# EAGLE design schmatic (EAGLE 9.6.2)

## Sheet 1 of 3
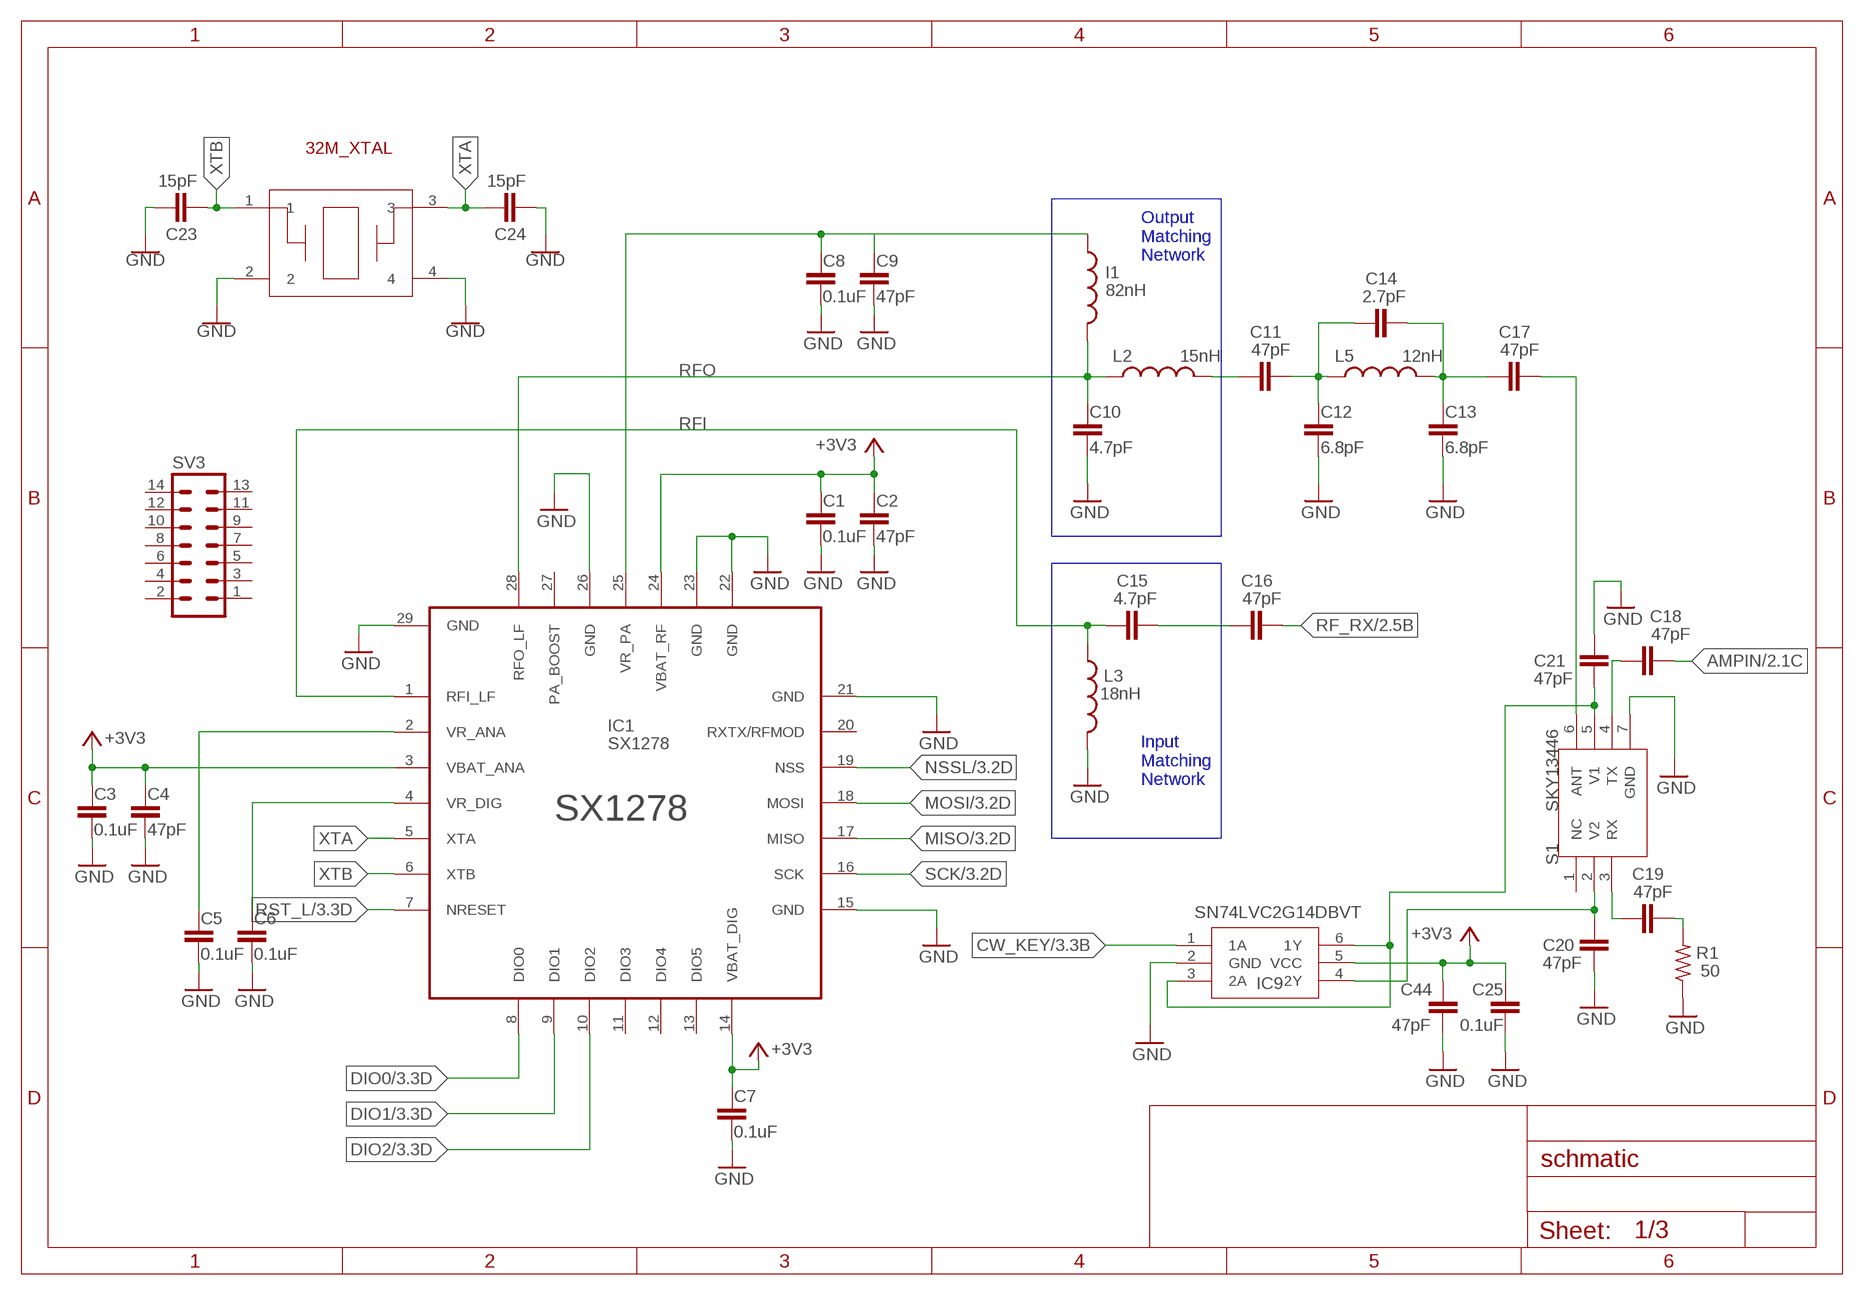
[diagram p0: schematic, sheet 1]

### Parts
C1  0.1uF  CAPACITOR  [M(1005)_US(0402)]
C2  47pF  CAPACITOR  [M(1005)_US(0402)]
C3  0.1uF  CAPACITOR  [M(1005)_US(0402)]
C4  47pF  CAPACITOR  [M(1005)_US(0402)]
C5  0.1uF  CAPACITOR  [M(1005)_US(0402)]
C6  0.1uF  CAPACITOR  [M(1005)_US(0402)]
C7  0.1uF  CAPACITOR  [M(1005)_US(0402)]
C8  0.1uF  CAPACITOR  [M(1005)_US(0402)]
C9  47pF  CAPACITOR  [M(1005)_US(0402)]
C10  4.7pF  CAPACITOR  [M(1005)_US(0402)]
C11  47pF  CAPACITOR  [M(1005)_US(0402)]
C12  6.8pF  CAPACITOR  [M(1005)_US(0402)]
C13  6.8pF  CAPACITOR  [M(1005)_US(0402)]
C14  2.7pF  CAPACITOR  [M(1005)_US(0402)]
C15  4.7pF  CAPACITOR  [M(1005)_US(0402)]
C16  47pF  CAPACITOR  [M(1005)_US(0402)]
C17  47pF  CAPACITOR  [M(1005)_US(0402)]
C18  47pF  CAPACITOR  [M(1005)_US(0402)]
C19  47pF  CAPACITOR  [M(1005)_US(0402)]
C20  47pF  CAPACITOR  [M(1005)_US(0402)]
C21  47pF  CAPACITOR  [M(1005)_US(0402)]
C23  15pF  CAP_(M1005)_0402  [CAP_(M1005)_0402]
C24  15pF  CAP_(M1005)_0402  [CAP_(M1005)_0402]
C25  0.1uF  CAPACITOR  [M(1005)_US(0402)]
C44  47pF  CAPACITOR  [M(1005)_US(0402)]
I1  82nH  INDUCTOR1608  [M(1608)_US(0603)]
IC1  SX1278  [SX1278]
IC9  SN74LVC2G14DBVT  SN74LVC2G34DBVR  [SOT-23-6]
L2  15nH  INDUCTOR  [M(1005)_US(0402)]
L3  18nH  INDUCTOR  [M(1005)_US(0402)]
L5  12nH  INDUCTOR  [M(1005)_US(0402)]
Q1  NX2520SA-32MHZ  [NX2520SA]
R1  50  RESISTOR1608  [M(1608)_US(0603)]
S1  SKY13446  [SKY13446]
SV3  ML14  [ML14]

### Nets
+3V1: C5.1 IC1.2(VR_ANA)
+3V2: C6.1 IC1.4(VR_DIG)
+3V3: C1.1 C2.1 C3.1 C4.1 C7.1 C25.1 C44.1 IC1.3(VBAT_ANA) IC1.14(VBAT_DIG) IC1.24(VBAT_RF) IC9.5(VCC) ; also sheet 2,3
+3V4: C8.1 C9.1 I1.1 IC1.25(VR_PA)
AMPIN: C18.2 ; also sheet 2
CW_KEY: IC9.1(1A) ; also sheet 3
DIO0: IC1.8(DIO0) ; also sheet 3
DIO1: IC1.9(DIO1) ; also sheet 3
DIO2: IC1.10(DIO2) ; also sheet 3
GND: C1.2 C2.2 C3.2 C4.2 C5.2 C6.2 C7.2 C8.2 C9.2 C10.2 C12.2 C13.2 C20.1 C21.2 C23.1 C24.2 C25.2 C44.2 IC1.15(GND) IC1.21(GND) IC1.22(GND) IC1.23(GND) IC1.26(GND) IC1.29(GND) IC9.2(GND) L3.2 Q1.2 Q1.4 R1.1 S1.7(GND) ; also sheet 2,3
MISO: IC1.17(MISO) ; also sheet 3
MOSI: IC1.18(MOSI) ; also sheet 3
N$1: C11.1 L2.2
N$2: C11.2 C12.1 C14.1 L5.1
N$3: C13.1 C14.2 C17.1 L5.2
N$4: C17.2 S1.6(ANT)
N$5: C15.2 C16.1
N$6: C18.1 S1.4(TX)
N$7: C19.1 S1.3(RX)
N$8: C19.2 R1.2
N$11: C20.2 IC9.4(2Y) S1.2(V2)
N$27: C21.1 IC9.3(2A) IC9.6(1Y) S1.5(V1)
NSSL: IC1.19(NSS) ; also sheet 3
RF_RX: C16.2 ; also sheet 2
RFI: C15.1 IC1.1(RFI_LF) L3.1
RFO: C10.1 I1.2 IC1.28(RFO_LF) L2.1
RST_L: IC1.7(NRESET) ; also sheet 3
SCK: IC1.16(SCK) ; also sheet 3
XTA: C24.1 IC1.5(XTA) Q1.3
XTB: C23.2 IC1.6(XTB) Q1.1
Unconnected: IC1.11(DIO3) IC1.12(DIO4) IC1.13(DIO5) IC1.20(RXTX/RFMOD) IC1.27(PA_BOOST) S1.1(NC) SV3.1 SV3.2 SV3.3 SV3.4 SV3.5 SV3.6 SV3.7 SV3.8 SV3.9 SV3.10 SV3.11 SV3.12 SV3.13 SV3.14

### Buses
B$1
B$2

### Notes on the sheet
- 32M_XTAL
- Output
  Matching
  Network
- Input
  Matching
  Network

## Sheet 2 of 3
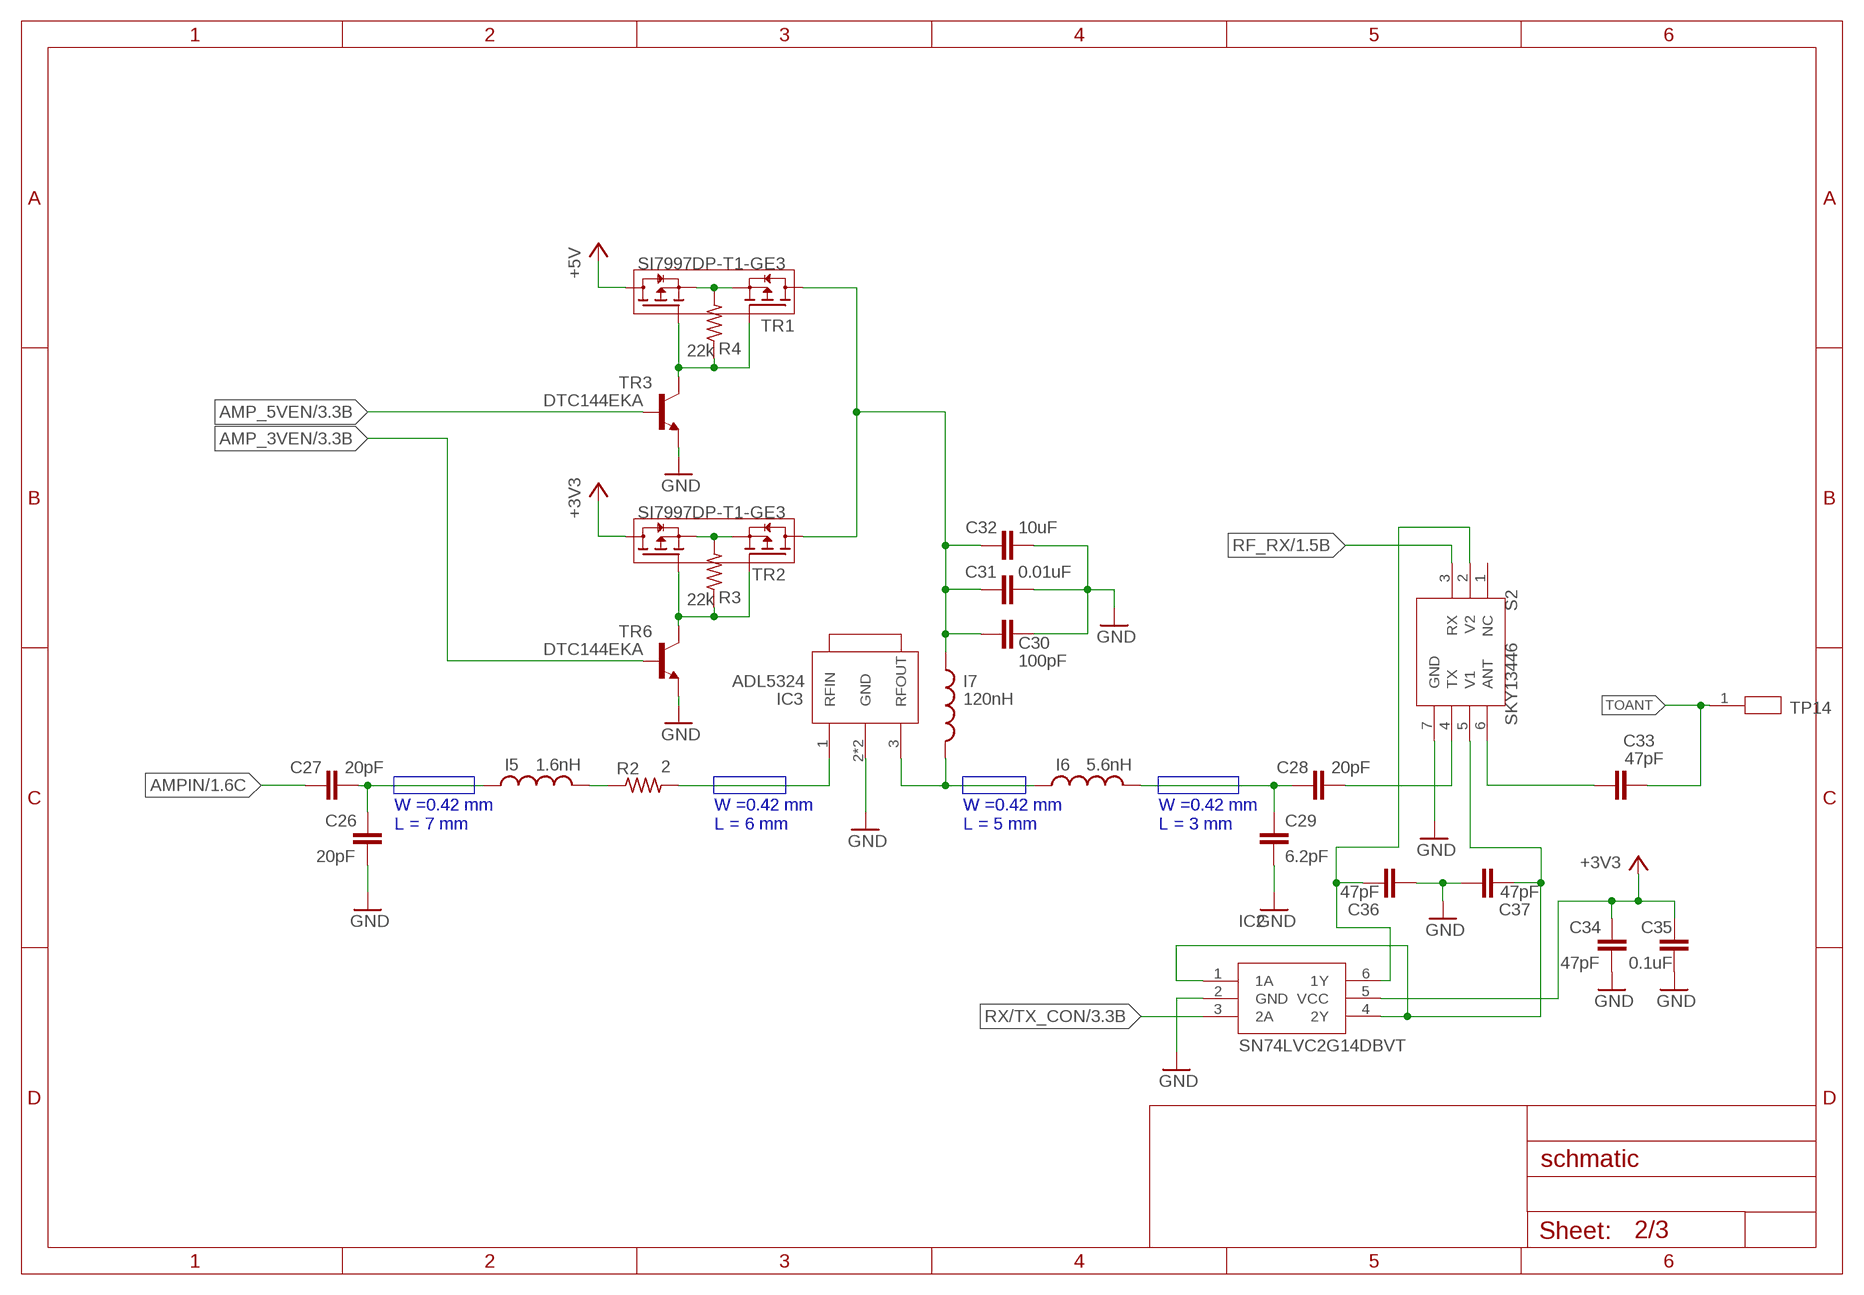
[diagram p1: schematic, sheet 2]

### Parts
C26  20pF  CAPACITOR  [M(1005)_US(0402)]
C27  20pF  CAPACITOR  [M(1005)_US(0402)]
C28  20pF  CAPACITOR  [M(1005)_US(0402)]
C29  6.2pF  CAPACITOR  [M(1005)_US(0402)]
C30  100pF  CAPACITOR  [M(1005)_US(0402)]
C31  0.01uF  CAPACITOR  [M(1005)_US(0402)]
C32  10uF  CAPACITOR1608  [M(1608)_US(0603)]
C33  47pF  CAPACITOR  [M(1005)_US(0402)]
C34  47pF  CAPACITOR  [M(1005)_US(0402)]
C35  0.1uF  CAPACITOR  [M(1005)_US(0402)]
C36  47pF  CAPACITOR  [M(1005)_US(0402)]
C37  47pF  CAPACITOR  [M(1005)_US(0402)]
I5  1.6nH  INDUCTOR  [M(1005)_US(0402)]
I6  5.6nH  INDUCTOR  [M(1005)_US(0402)]
I7  120nH  INDUCTOR2012  [M(2012)_US(0805)]
IC2  SN74LVC2G14DBVT  SN74LVC2G34DBVR  [SOT-23-6]
IC3  ADL5324  [ADL5324]
R2  2  RESISTOR1608  [M(1608)_US(0603)]
R3  22k  RESISTOR1608  [M(1608)_US(0603)]
R4  22k  RESISTOR1608  [M(1608)_US(0603)]
S2  SKY13446  [SKY13446]
TP14  TEST_POINT  [TEST_POINT_1.5MM]
TR1  SI7997DP-T1-GE3  [SI7997DP-T1-GE3]
TR2  SI7997DP-T1-GE3  [SI7997DP-T1-GE3]
TR3  DTC144EKA  [SOT346-R]
TR6  DTC144EKA  [SOT346-R]

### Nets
+3V3: C34.1 C35.1 IC2.5(VCC) TR2.7(D1) TR2.8(D1) TR2.10(D1) ; also sheet 1,3
+3V5: C30.1
+5V: TR1.7(D1) TR1.8(D1) TR1.10(D1) ; also sheet 3
AMP_3VEN: TR6.2(B) ; also sheet 3
AMP_5VEN: TR3.2(B) ; also sheet 3
AMPIN: C27.1 ; also sheet 1
AMPPWR: C30.2 C31.2 C32.1 I7.1 TR1.5(D2) TR1.6(D2) TR1.9(D2) TR2.5(D2) TR2.6(D2) TR2.9(D2)
GND: C26.2 C29.2 C31.1 C32.2 C34.2 C35.2 C36.1 C37.2 IC2.2(GND) IC3.2(GND) IC3.4(GND) S2.7(GND) TR3.1(E) TR6.1(E) ; also sheet 1,3
N$9: C26.1 C27.2 I5.1
N$10: C37.1 IC2.1(1A) IC2.4(2Y) S2.5(V1)
N$12: I5.2 R2.1
N$13: IC3.1(RFIN) R2.2
N$14: I6.1 I7.2 IC3.3(RFOUT)
N$15: C28.1 C29.1 I6.2
N$16: C28.2 S2.4(TX)
N$17: C33.1 S2.6(ANT)
N$18: R4.2 TR1.1(S1) TR1.3(S2)
N$19: R3.2 TR2.1(S1) TR2.3(S2)
N$20: C36.2 IC2.6(1Y) S2.2(V2)
N$22: R4.1 TR1.2(G1) TR1.4(G2) TR3.3(C)
N$23: R3.1 TR2.2(G1) TR2.4(G2) TR6.3(C)
RF_RX: S2.3(RX) ; also sheet 1
RX/TX_CON: IC2.3(2A) ; also sheet 3
TOANT: C33.2 TP14.1
Unconnected: S2.1(NC)

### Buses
B$3
B$4
B$5
B$6

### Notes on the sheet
- W =0.42 mm
  L = 7 mm
- W =0.42 mm
  L = 6 mm
- W =0.42 mm
  L = 5 mm
- W =0.42 mm
  L = 3 mm

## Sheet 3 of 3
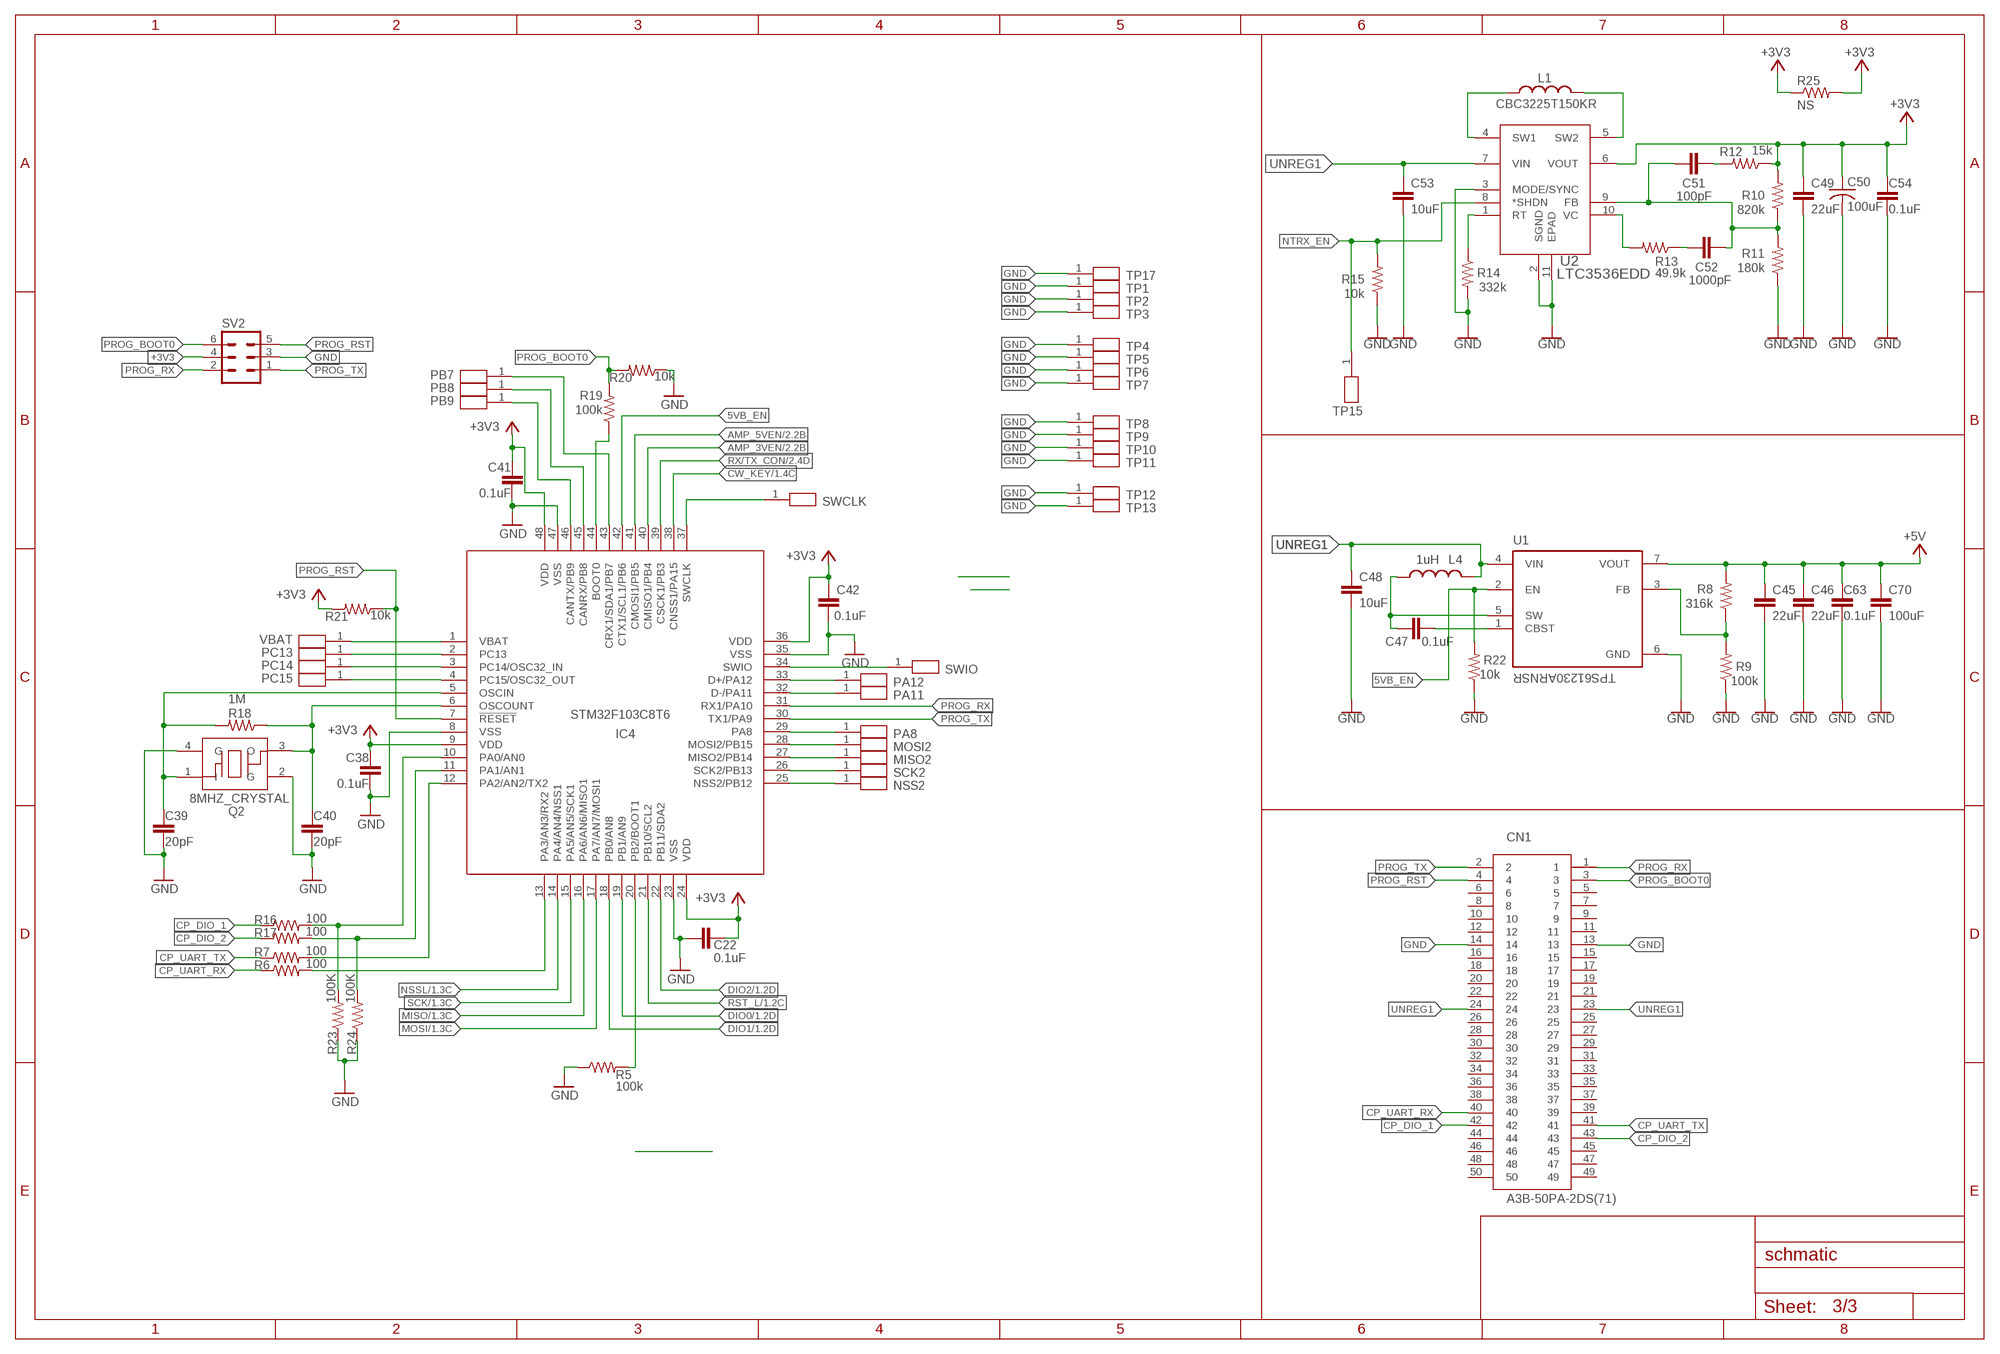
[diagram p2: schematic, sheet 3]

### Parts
C22  0.1uF  CAPACITOR  [M(1005)_US(0402)]
C38  0.1uF  CAPACITOR  [M(1005)_US(0402)]
C39  20pF  CAPACITOR  [M(1005)_US(0402)]
C40  20pF  CAPACITOR  [M(1005)_US(0402)]
C41  0.1uF  CAPACITOR  [M(1005)_US(0402)]
C42  0.1uF  CAPACITOR  [M(1005)_US(0402)]
C45  22uF  CAPACITOR1608  [M(1608)_US(0603)]
C46  22uF  CAPACITOR1608  [M(1608)_US(0603)]
C47  0.1uF  CAPACITOR  [M(1005)_US(0402)]
C48  10uF  CAPACITOR1608  [M(1608)_US(0603)]
C49  22uF  CAPACITOR1608  [M(1608)_US(0603)]
C50  100uF  C-USC1210  [C1210]
C51  100pF  CAPACITOR  [M(1005)_US(0402)]
C52  1000pF  CAPACITOR  [M(1005)_US(0402)]
C53  10uF  CAPACITOR1608  [M(1608)_US(0603)]
C54  0.1uF  CAPACITOR  [M(1005)_US(0402)]
C63  0.1uF  CAPACITOR  [M(1005)_US(0402)]
C70  100uF  CAPACITOR2012  [M(2012)_US(0805)]
CN1  A3B-50PA-2DS(71)  [A3B-50PA-2DS(71)]
IC4  STM32F103C8T6  [STM32F103C8T6]
L1  CBC3225T150KR  INDUCTOR3225  [M(3225)_US(1210)]
L4  1uH  AMDLA3020S-1R5MT  [AMDLA3020S-1R5MT]
MISO2  TEST_POINT  [TEST_POINT_1.5MM]
MOSI2  TEST_POINT  [TEST_POINT_1.5MM]
NSS2  TEST_POINT  [TEST_POINT_1.5MM]
PA8  TEST_POINT  [TEST_POINT_1.5MM]
PA11  TEST_POINT  [TEST_POINT_1.5MM]
PA12  TEST_POINT  [TEST_POINT_1.5MM]
PB7  TEST_POINT  [TEST_POINT_1.5MM]
PB8  TEST_POINT  [TEST_POINT_1.5MM]
PB9  TEST_POINT  [TEST_POINT_1.5MM]
PC13  TEST_POINT  [TEST_POINT_1.5MM]
PC14  TEST_POINT  [TEST_POINT_1.5MM]
PC15  TEST_POINT  [TEST_POINT_1.5MM]
Q2  8MHZ_CRYSTAL  [ECS-80-18-30B-JEM-TR]
R5  100k  RESISTOR  [M(1005)_US(0402)]
R6  100  RESISTOR  [M(1005)_US(0402)]
R7  100  RESISTOR  [M(1005)_US(0402)]
R8  316k  RESISTOR1608  [M(1608)_US(0603)]
R9  100k  RESISTOR1608  [M(1608)_US(0603)]
R10  820k  RESISTOR1608  [M(1608)_US(0603)]
R11  180k  RESISTOR1608  [M(1608)_US(0603)]
R12  15k  RESISTOR1608  [M(1608)_US(0603)]
R13  49.9k  RESISTOR1608  [M(1608)_US(0603)]
R14  332k  RESISTOR1608  [M(1608)_US(0603)]
R15  10k  RESISTOR  [M(1005)_US(0402)]
R16  100  RESISTOR  [M(1005)_US(0402)]
R17  100  RESISTOR  [M(1005)_US(0402)]
R18  1M  RESISTOR1608  [M(1608)_US(0603)]
R19  100k  RESISTOR  [M(1005)_US(0402)]
R20  10k  RESISTOR  [M(1005)_US(0402)]
R21  10k  RESISTOR  [M(1005)_US(0402)]
R22  10k  RESISTOR  [M(1005)_US(0402)]
R23  100K  RESISTOR  [M(1005)_US(0402)]
R24  100K  RESISTOR  [M(1005)_US(0402)]
R25  NS  RESISTOR2012  [M(2012)_US(0805)]
SCK2  TEST_POINT  [TEST_POINT_1.5MM]
SV2  MA03-2  [MA03-2]
SWCLK  TEST_POINT  [TEST_POINT_1.5MM]
SWIO  TEST_POINT  [TEST_POINT_1.5MM]
TP1  TEST_POINT  [TEST_POINT_1.5MM]
TP2  TEST_POINT  [TEST_POINT_1.5MM]
TP3  TEST_POINT  [TEST_POINT_1.5MM]
TP4  TEST_POINT  [TEST_POINT_1.5MM]
TP5  TEST_POINT  [TEST_POINT_1.5MM]
TP6  TEST_POINT  [TEST_POINT_1.5MM]
TP7  TEST_POINT  [TEST_POINT_1.5MM]
TP8  TEST_POINT  [TEST_POINT_1.5MM]
TP9  TEST_POINT  [TEST_POINT_1.5MM]
TP10  TEST_POINT  [TEST_POINT_1.5MM]
TP11  TEST_POINT  [TEST_POINT_1.5MM]
TP12  TEST_POINT  [TEST_POINT_1.5MM]
TP13  TEST_POINT  [TEST_POINT_1.5MM]
TP15  TEST_POINT  [TEST_POINT_1.5MM]
TP17  TEST_POINT  [TEST_POINT_1.5MM]
U1  TPS61230ARNSR  [IC_TPS61230ARNSR]
U2  LTC3536EDD  LTC3536EDD#TRPBF  [DFN-10_DD]
VBAT  TEST_POINT  [TEST_POINT_1.5MM]

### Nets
5VB_EN: IC4.42(CTX1/SCL1/PB6) R22.2 U1.2(EN)
+3V3: C22.1 C38.1 C41.1 C42.1 C49.1 C50.1 C54.1 IC4.9(VDD) IC4.24(VDD) IC4.36(VDD) IC4.48(VDD) R10.2 R12.1 R21.2 R25.1 R25.2 SV2.4 U2.6(VOUT) ; also sheet 1,2
+5V: C45.1 C46.1 C63.1 C70.1 R8.2 U1.7(VOUT) ; also sheet 2
AMP_3VEN: IC4.40(CMISO1/PB4) ; also sheet 2
AMP_5VEN: IC4.41(CMOSI1/PB5) ; also sheet 2
C_UART_RX: IC4.13(PA3/AN3/RX2) R6.2
C_UART_TX: IC4.12(PA2/AN2/TX2) R7.2
CP_DIO_1: CN1.42 R16.1
CP_DIO_2: CN1.43 R17.1
CP_UART_RX: CN1.40 R6.1
CP_UART_TX: CN1.41 R7.1
CW_KEY: IC4.38(CNSS1/PA15) ; also sheet 1
DIO0: IC4.19(PB1/AN9) ; also sheet 1
DIO1: IC4.18(PB0/AN8) ; also sheet 1
DIO2: IC4.22(PB11/SDA2) ; also sheet 1
GND: C22.2 C38.2 C39.2 C40.2 C41.2 C42.2 C45.2 C46.2 C48.2 C49.2 C50.2 C53.2 C54.2 C63.2 C70.2 CN1.13 CN1.14 IC4.8(VSS) IC4.23(VSS) IC4.35(VSS) IC4.47(VSS) Q2.2(G) Q2.4(G) R5.1 R9.1 R11.1 R14.2 R15.1 R20.1 R22.1 R23.1 R24.1 SV2.3 TP1.1 TP2.1 TP3.1 TP4.1 TP5.1 TP6.1 TP7.1 TP8.1 TP9.1 TP10.1 TP11.1 TP12.1 TP13.1 TP17.1 U1.6(GND) U2.2(SGND) U2.3(MODE/SYNC) U2.11(EPAD) ; also sheet 1,2
MISO: IC4.16(PA6/AN6/MISO1) ; also sheet 1
MOSI: IC4.17(PA7/AN7/MOSI1) ; also sheet 1
N$24: IC4.10(PA0/AN0) R16.2 R23.2
N$25: IC4.20(PB2/BOOT1) R5.2
N$26: IC4.11(PA1/AN1) R17.2 R24.2
N$28: C39.1 IC4.5(OSCIN) Q2.1(I) R18.2
N$29: C40.1 IC4.6(OSCOUNT) Q2.3(O) R18.1
N$30: L1.1 U2.4(SW1)
N$31: R8.1 R9.2 U1.3(FB)
N$32: C47.1 L4.1 U1.5(SW)
N$33: L1.2 U2.5(SW2)
N$34: C47.2 U1.1(CBST)
N$35: IC4.1(VBAT) VBAT.1
N$36: C51.2 R12.2
N$37: C51.1 C52.2 R10.1 R11.2 U2.9(FB)
N$38: IC4.44(BOOT0) R19.1
N$39: C52.1 R13.1
N$40: R13.2 U2.10(VC)
N$41: R14.1 U2.1(RT)
N$42: IC4.4(PC15/OSC32_OUT) PC15.1
N$44: IC4.3(PC14/OSC32_IN) PC14.1
N$45: IC4.2(PC13) PC13.1
N$46: IC4.27(MISO2/PB14) MISO2.1
N$47: IC4.28(MOSI2/PB15) MOSI2.1
N$48: IC4.33(D+/PA12) PA12.1
N$49: IC4.32(D-/PA11) PA11.1
N$50: IC4.29(PA8) PA8.1
N$68: IC4.26(SCK2/PB13) SCK2.1
N$69: IC4.25(NSS2/PB12) NSS2.1
NSSL: IC4.14(PA4/AN4/NSS1) ; also sheet 1
NTRX_EN: R15.2 TP15.1 U2.8(*SHDN)
PB7: IC4.43(CRX1/SDA1/PB7) PB7.1
PB8: IC4.45(CANRX/PB8) PB8.1
PB9: IC4.46(CANTX/PB9) PB9.1
PROG_BOOT0: CN1.3 R19.2 R20.2 SV2.6
PROG_RST: CN1.4 IC4.7(!RESET) R21.1 SV2.5
PROG_RX: CN1.1 IC4.31(RX1/PA10) SV2.2
PROG_TX: CN1.2 IC4.30(TX1/PA9) SV2.1
RST_L: IC4.21(PB10/SCL2) ; also sheet 1
RX/TX_CON: IC4.39(CSCK1/PB3) ; also sheet 2
SCK: IC4.15(PA5/AN5/SCK1) ; also sheet 1
SWCLK: IC4.37(SWCLK) SWCLK.1
SWIO: IC4.34(SWIO) SWIO.1
UNREG1: C48.1 C53.1 CN1.23 CN1.24 L4.2 U1.4(VIN) U2.7(VIN)
Unconnected: CN1.5 CN1.6 CN1.7 CN1.8 CN1.9 CN1.10 CN1.11 CN1.12 CN1.15 CN1.16 CN1.17 CN1.18 CN1.19 CN1.20 CN1.21 CN1.22 CN1.25 CN1.26 CN1.27 CN1.28 CN1.29 CN1.30 CN1.31 CN1.32 CN1.33 CN1.34 CN1.35 CN1.36 CN1.37 CN1.38 CN1.39 CN1.44 CN1.45 CN1.46 CN1.47 CN1.48 CN1.49 CN1.50

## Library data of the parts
C1-C22 C25-C42 C44-C49 C51-C54 C63 C70 = Tharindu_lib:CAPACITOR
C23 C24 = Tharindu:CAP_(M1005)_0402
C50 = adafruit:C-US: CAPACITOR, American symbol
CN1 = Tharindu1:A3B-50PA-2DS(71)
I1 I5-I7 L1-L3 L5 = Tharindu_lib:INDUCTOR
IC1 = Tharindu:SX1278
IC2 IC9 = Tharindu:SN74LVC2G34DBVR
IC3 = Tharindu:ADL5324
IC4 = Tharindu:STM32F103C8T6
L4 = Tharindu:AMDLA3020S-1R5MT
MISO2 MOSI2 NSS2 PA8 PA11 PA12 PB7-PB9 PC13-PC15 SCK2 SWCLK SWIO TP1-TP15 TP17 VBAT = Tharindu:TEST_POINT
Q1 = Tharindu:NX2520SA-32MHZ
Q2 = Tharindu:8MHZ_CRYSTAL
R1-R25 = Tharindu_lib:RESISTOR
S1 S2 = Tharindu:SKY13446
SV2 = con-lstb:MA03-2: PIN HEADER; OC_FARNELL: unknown; OC_NEWARK: unknown
SV3 = con-ml:ML14: HARTING; OC_FARNELL: unknown; OC_NEWARK: unknown
TR1 TR2 = Tharindu:SI7997DP-T1-GE3
TR3 TR6 = BIRDS3_CAM_MSN:DTC144EKA
U1 = TPS61230ARNSR:TPS61230ARNSR: Boost Switching Regulator IC Positive Adjustable 2.5V 1 Output 6A (Switch) 7-VFQFN Check availability; AVAILABILITY: In Stock; DESCRIPTION: 5-V/6-A High Efficiency Step-Up Converter in 2.0-mm x 2.0-mm QFN Package; MF: Texas Instruments; MP: TPS61230ARNSR; PACKAGE: VQFN-HR-7 Texas Instruments; PRICE: None; PURCHASE-URL: https://pricing.snapeda.com/search/part/TPS61230ARNSR/?ref=eda
U2 = LTC3536EDD_TRPBF:LTC3536EDD#TRPBF: Check availability; AVAILABILITY: In Stock; DESCRIPTION: 1A Low Noise, Buck-Boost DC/DC Converter; MF: Analog Devices; MP: LTC3536EDD#TRPBF; PACKAGE: DFN -10 Analog Devices; PRICE: None; PURCHASE-URL: https://pricing.snapeda.com/search/part/LTC3536EDD#TRPBF/?ref=eda

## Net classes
0 default: width 0.203 mm, drill 0.33 mm, clearance 0.203 mm
2 gnd: width 0.305 mm, drill 0.33 mm, clearance 0.203 mm
3 power usb: width 0.508 mm, drill 0.33 mm, clearance 0.203 mm

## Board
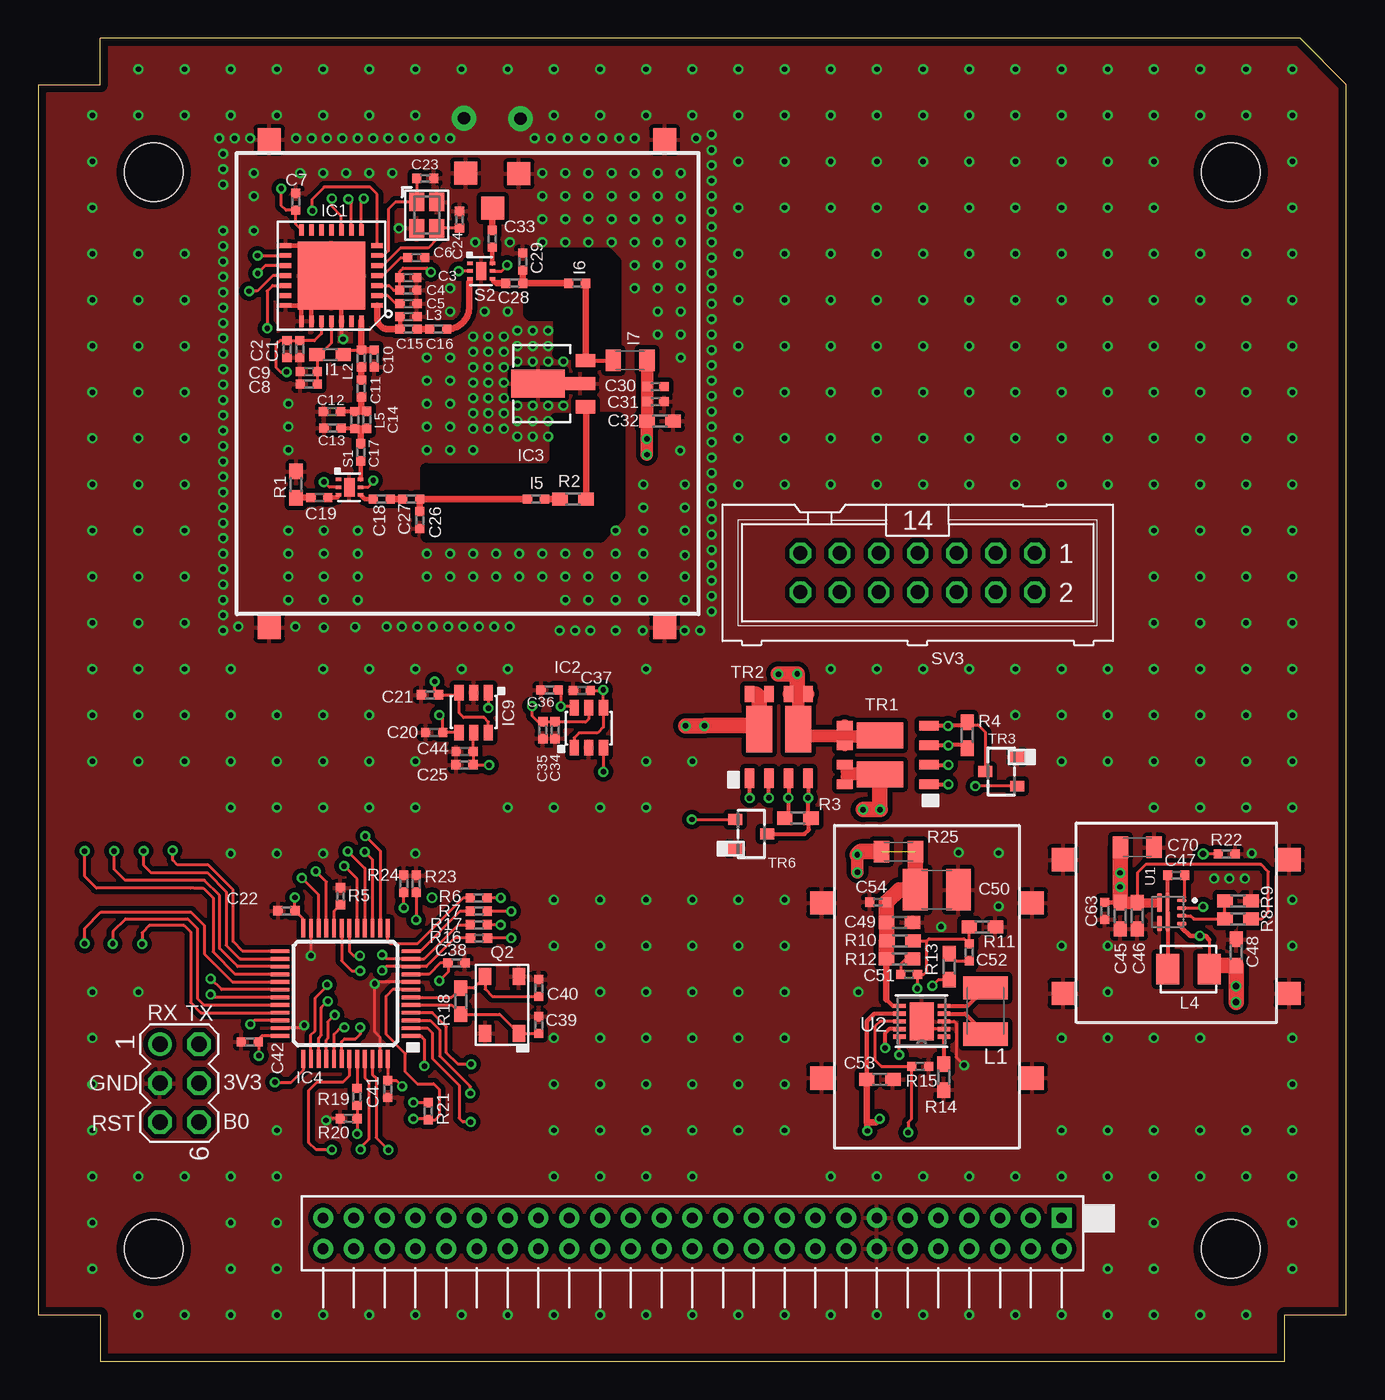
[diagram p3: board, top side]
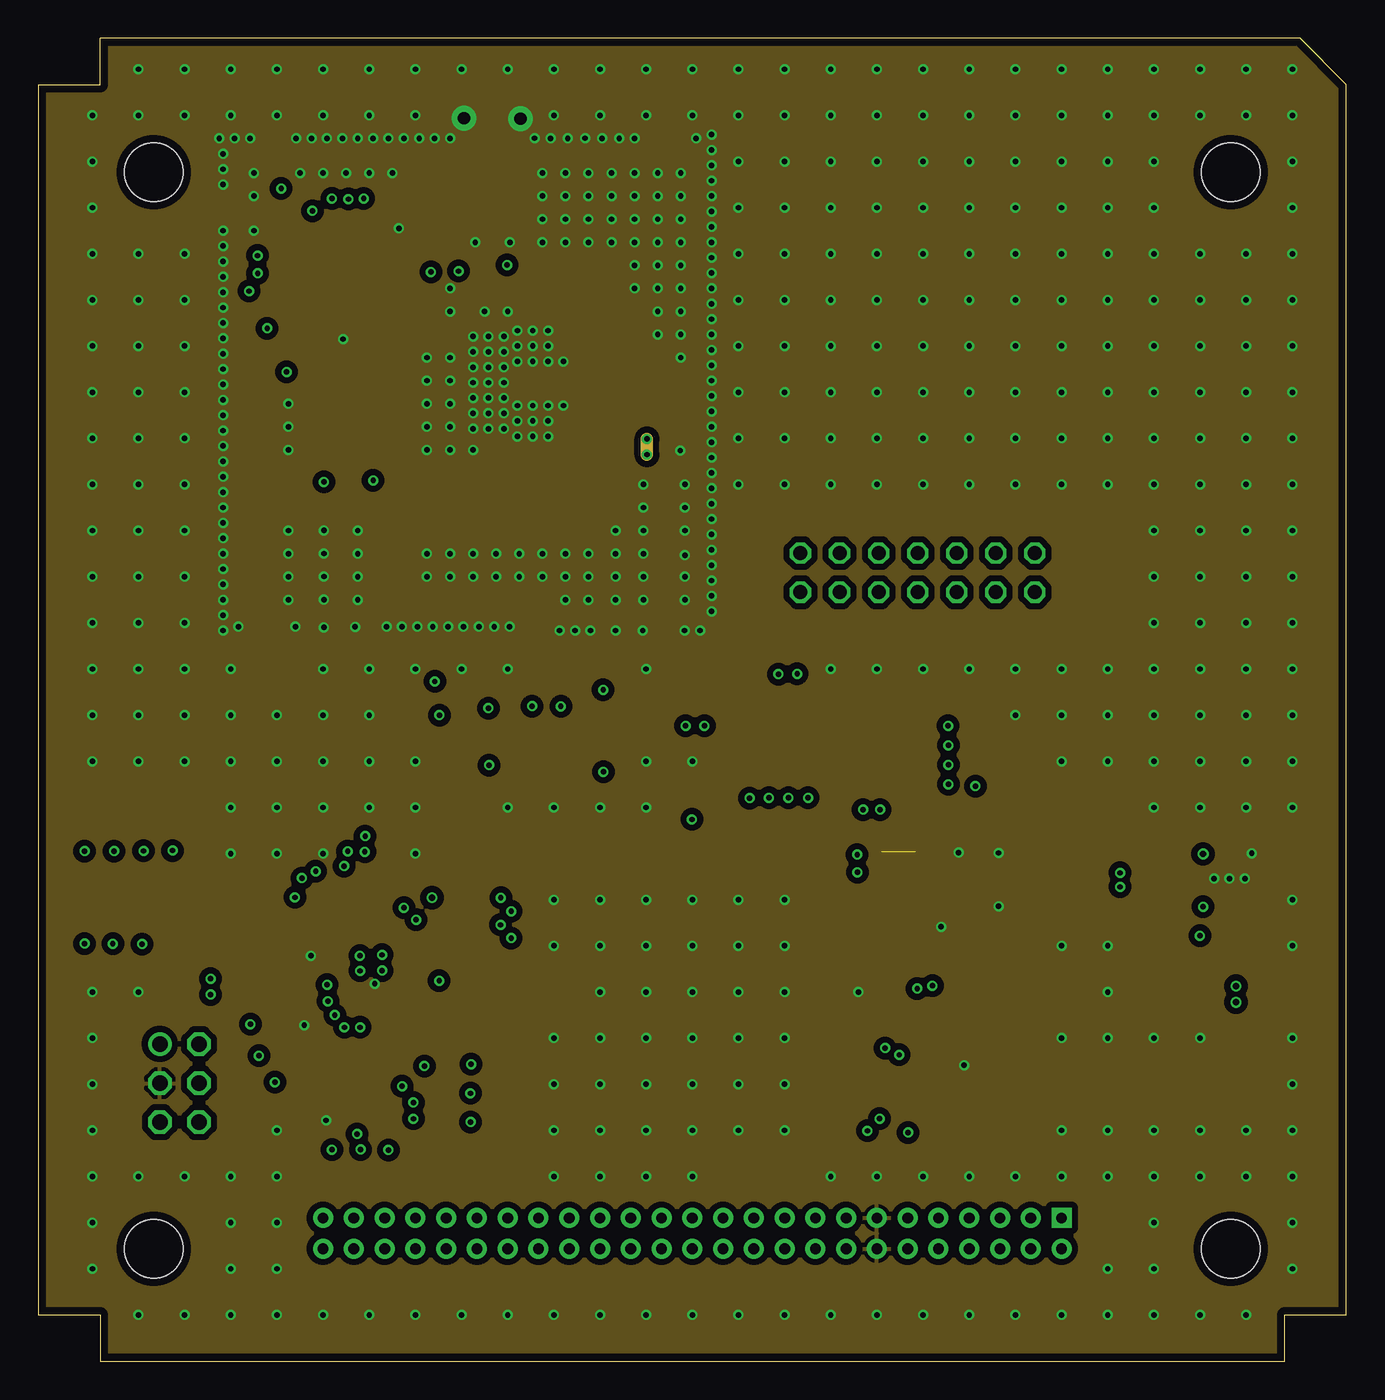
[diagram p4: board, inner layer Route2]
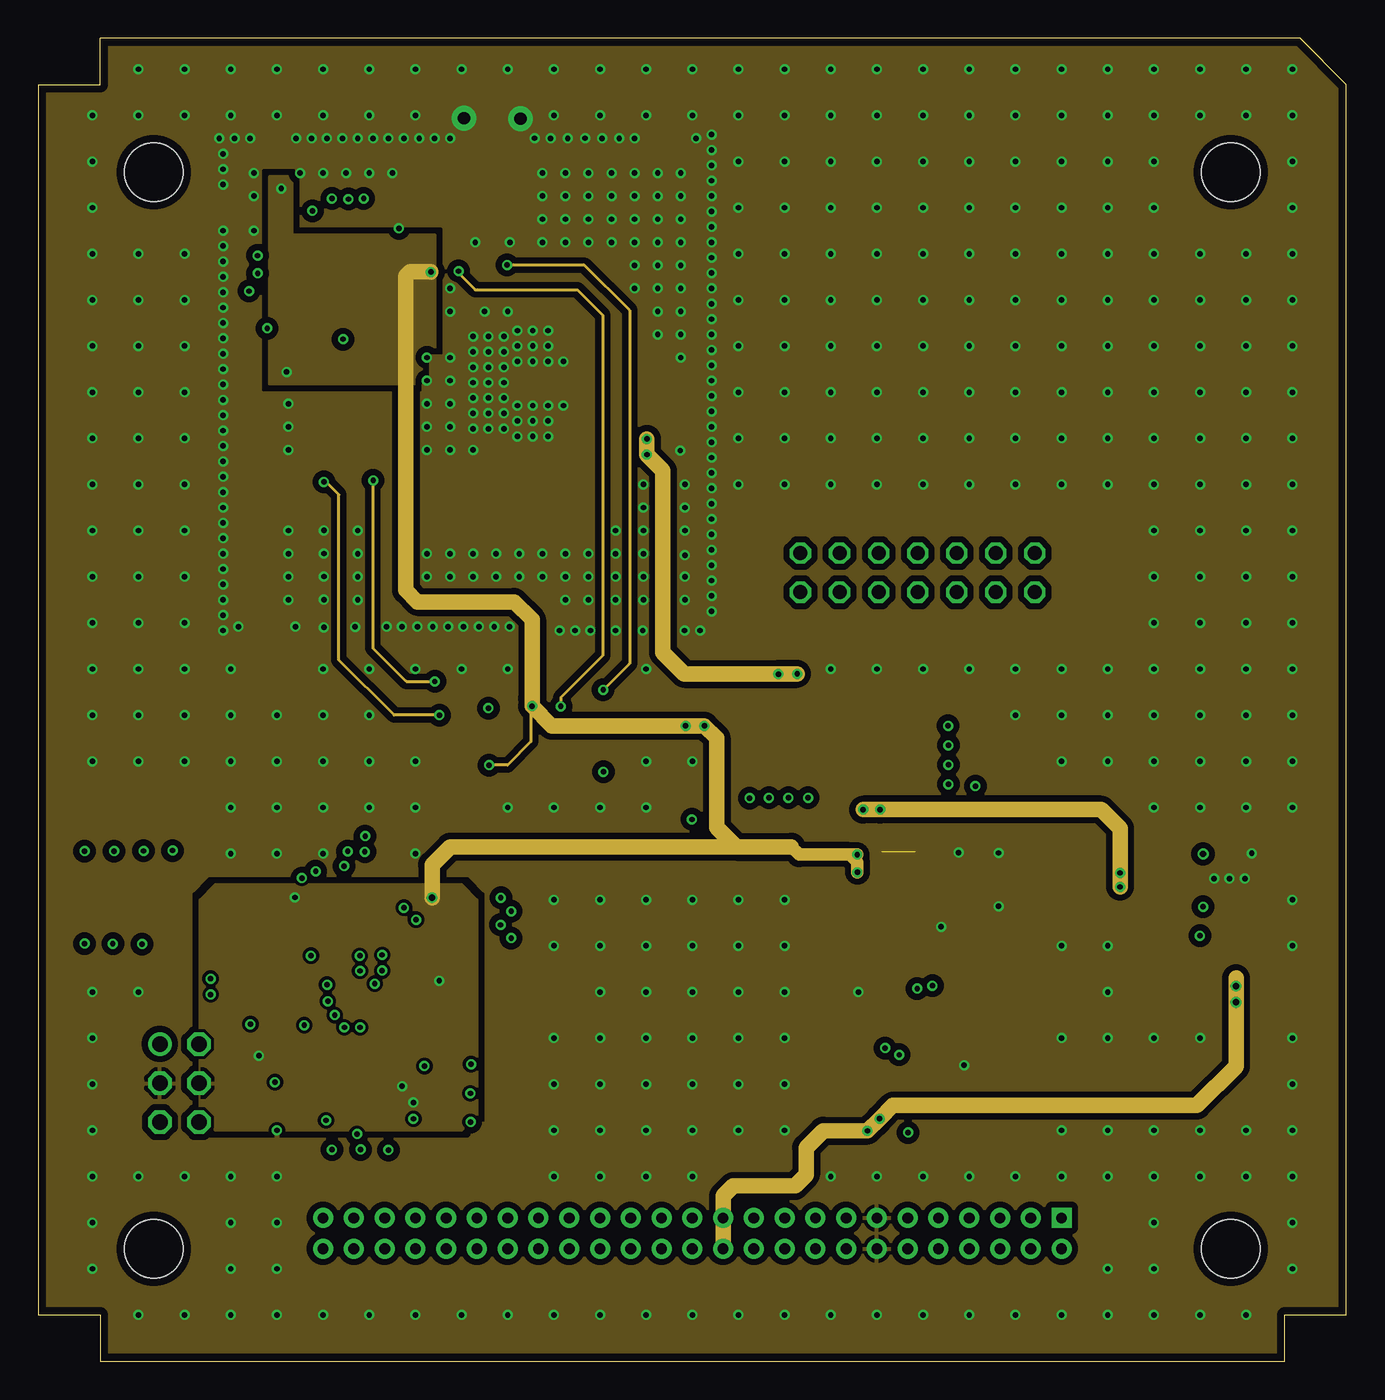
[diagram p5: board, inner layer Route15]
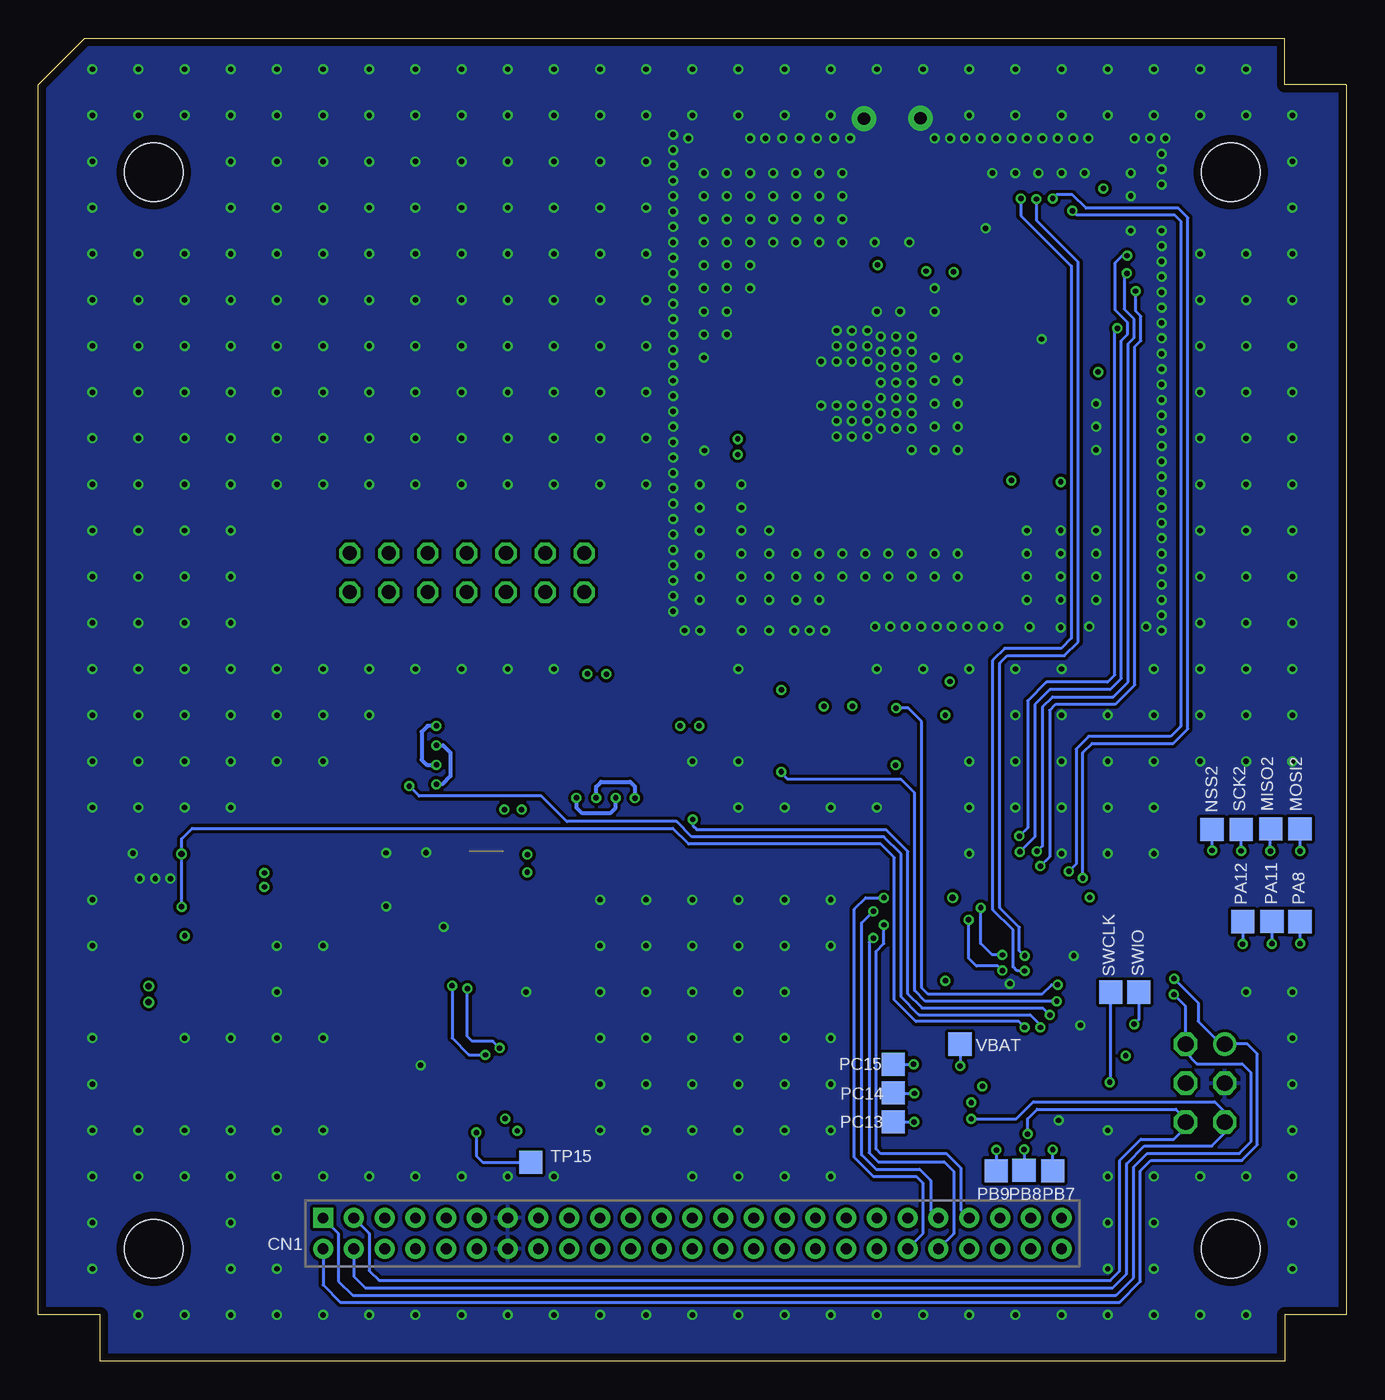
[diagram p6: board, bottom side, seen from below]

Size 85 x 86 mm. Coordinates in mm from the lower left corner, seen from the top.
Outline: 4,0 81,0 81,3 85,3 85,83 82,86 4,86 4,83 0,83 0,3 4,3 4,0
Copper layers (1+2*15+16): Top 0.018mm / dielectric 0.25mm / Route2 0.035mm / dielectric 1mm / Route15 0.035mm / dielectric 0.25mm / Bottom 0.018mm
Design rules "pban_5mil-l4": minimum track width 5mil, minimum drill 0.3mm, track to track 5mil, track to pad 0.229mm, pad to pad 5mil, via to via 5mil, smd to smd 5mil, copper to edge 0.5mm, drill to drill 0.5mm, minimum pad ring 0.15mm, minimum via ring 0.15mm, stop-mask expansion 4mil, vias tented up to drill 0.35mm, thermal gap 10mil
Holes 3.8 mm at 77.5,7.3 7.5,7.3 7.5,77.3 77.5,77.3
tRestrict: 19 lines

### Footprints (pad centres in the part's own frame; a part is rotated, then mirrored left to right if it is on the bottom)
M(1005)_US(0402) = smd 0.6 x 0.6: 1 -0.55,0; 2 0.55,0
CAP_(M1005)_0402 = smd 0.6 x 0.6: 1 -0.55,0; 2 0.55,0
M(1608)_US(0603) = smd 1 x 0.85: 1 -0.85,0; 2 0.85,0
C1210 = smd 1.6 x 2.7: 1 -1.4,0; 2 1.4,0
M(2012)_US(0805) = smd 1 x 1.4: 1 -1.1,0; 2 1.1,0
A3B-50PA-2DS(71) = drill 0.7 pad 1.3 square: 1 0,2 | drill 0.7 pad 1.3: 2 0,0; 3 2,2; 4 2,0; 5 4,2; 6 4,0; 7 6,2; 8 6,0; 9 8,2; 10 8,0; 11 10,2; 12 10,0; 13 12,2; 14 12,0; 15 14,2; 16 14,0; 17 16,2; 18 16,0; 19 18,2; 20 18,0; 21 20,2; 22 20,0; 23 22,2; 24 22,0; 25 24,2; 26 24,0; 27 26,2; 28 26,0; 29 28,2; 30 28,0; 31 30,2; 32 30,0; 33 32,2; 34 32,0; 35 34,2; 36 34,0; 37 36,2; 38 36,0; 39 38,2; 40 38,0; 41 40,2; 42 40,0; 43 42,2; 44 42,0; 45 44,2; 46 44,0; 47 46,2; 48 46,0; 49 48,2; 50 48,0
SX1278 = smd 0.75 x 0.3: 1 -2.975,1.95; 2 -2.975,1.3; 3 -2.975,0.65; 4 -2.975,0; 5 -2.975,-0.65; 6 -2.975,-1.3; 7 -2.975,-1.95; 15 2.975,-1.95; 16 2.975,-1.3; 17 2.975,-0.65; 18 2.975,0; 19 2.975,0.65; 20 2.975,1.3; 21 2.975,1.95 | smd 0.3 x 0.75: 8 -1.95,-2.975; 9 -1.3,-2.975; 10 -0.65,-2.975; 11 0,-2.975; 12 0.65,-2.975; 13 1.3,-2.975; 14 1.95,-2.975; 22 1.95,2.975; 23 1.3,2.975; 24 0.65,2.975; 25 0,2.975; 26 -0.65,2.975; 27 -1.3,2.975; 28 -1.95,2.975 | smd 4.4 x 4.4: 29 0,0
SOT-23-6 = smd 0.6 x 1: 1 -0.95,-1.3; 2 0,-1.3; 3 0.95,-1.3; 4 0.95,1.3; 5 0,1.3; 6 -0.95,1.3
ADL5324 = smd 0.86 x 1.27: 1 -1.5,0; 3 1.5,0 | smd 0.86 x 2: 2 0,0.365 | smd 1.8 x 3.48: 4 0,3.1
STM32F103C8T6 = smd 1.2 x 0.25: 1 -4.25,2.75; 2 -4.25,2.25; 3 -4.25,1.75; 4 -4.25,1.25; 5 -4.25,0.75; 6 -4.25,0.25; 7 -4.25,-0.25; 8 -4.25,-0.75; 9 -4.25,-1.25; 10 -4.25,-1.75; 11 -4.25,-2.25; 12 -4.25,-2.75; 25 4.25,-2.75; 26 4.25,-2.25; 27 4.25,-1.75; 28 4.25,-1.25; 29 4.25,-0.75; 30 4.25,-0.25; 31 4.25,0.25; 32 4.25,0.75; 33 4.25,1.25; 34 4.25,1.75; 35 4.25,2.25; 36 4.25,2.75 | smd 0.25 x 1.2: 13 -2.75,-4.25; 14 -2.25,-4.25; 15 -1.75,-4.25; 16 -1.25,-4.25; 17 -0.75,-4.25; 18 -0.25,-4.25; 19 0.25,-4.25; 20 0.75,-4.25; 21 1.25,-4.25; 22 1.75,-4.25; 23 2.25,-4.25; 24 2.75,-4.25; 37 2.75,4.25; 38 2.25,4.25; 39 1.75,4.25; 40 1.25,4.25; 41 0.75,4.25; 42 0.25,4.25; 43 -0.25,4.25; 44 -0.75,4.25; 45 -1.25,4.25; 46 -1.75,4.25; 47 -2.25,4.25; 48 -2.75,4.25
M(3225)_US(1210) = smd 1.5 x 2.9: 1 -1.5,0; 2 1.5,0
AMDLA3020S-1R5MT = smd 1.5 x 2: 1 -1.35,0; 2 1.35,0
TEST_POINT_1.5MM = smd 1.5 x 1.5: 1 0,0
NX2520SA = smd 1.2 x 1: 1 -0.85,-0.65; 2 0.85,-0.65; 3 0.85,0.65; 4 -0.85,0.65
ECS-80-18-30B-JEM-TR = smd 1.1 x 0.8: 1 -1.85,-1.1; 2 1.85,-1.1; 3 1.85,1.1; 4 -1.85,1.1
SKY13446 = smd 0.229 x 0.35: 1 0,0; 2 0.5,0; 3 1,0; 4 1,1.45; 5 0.5,1.45; 6 0,1.45 | smd 1.2 x 0.66: 7 0.5,0.725
MA03-2 = drill 1.016: 1 -2.54,-1.27 | drill 1.016 octagon: 2 -2.54,1.27; 3 0,-1.27; 4 0,1.27; 5 2.54,-1.27; 6 2.54,1.27
ML14 = drill 0.914 octagon: 1 -7.62,-1.27; 2 -7.62,1.27; 3 -5.08,-1.27; 4 -5.08,1.27; 5 -2.54,-1.27; 6 -2.54,1.27; 7 0,-1.27; 8 0,1.27; 9 2.54,-1.27; 10 2.54,1.27; 11 5.08,-1.27; 12 5.08,1.27; 13 7.62,-1.27; 14 7.62,1.27
SI7997DP-T1-GE3 = smd 1.27 x 0.61: 1 0,1.905; 2 0,0.635; 3 0,-0.635; 4 0,-1.905 | smd 1.02 x 0.61: 5 5.465,-1.905; 6 5.465,-0.635; 7 5.465,0.635; 8 5.465,1.905 | smd 3 x 1.7: 9 3.175,-1.27; 10 3.175,1.27
SOT346-R = smd 0.7 x 0.9: 1 0.95,-1.05; 2 -0.95,-1.05; 3 0,1.05
IC_TPS61230ARNSR = smd 0.25 x 0.6: 1 -0.75,0.9; 2 -0.25,0.9; 3 0.25,0.9; 4 0.75,0.9 | smd 2.5 x 0.279: 5 0,-0.015 | smd 1 x 0.33: 6 0.75,-0.54 | smd 1.219 x 0.33: 7 -0.6,-0.54
DFN-10_DD = smd 0.813 x 0.279: 1 -1.448,1; 2 -1.448,0.5; 3 -1.448,0; 4 -1.448,-0.5; 5 -1.448,-1; 6 1.448,-1; 7 1.448,-0.5; 8 1.448,0; 9 1.448,0.5; 10 1.448,1 | smd 1.575 x 2.489: 11 0,0

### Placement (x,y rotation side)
C1  16.99,65.8 270 top
C2  16.16,65.8 270 top
C3  24.04,70.44 0 top
C4  24.04,69.63 0 top
C5  24.05,68.76 0 top
C6  24.56,71.74 0 top
C7  16.72,75.38 90 top
C8  17.57,63.52 180 top
C9  17.57,64.34 180 top
C10  21.82,65.19 270 top
C11  20.99,63.24 270 top
C12  19.08,61.73 180 top
C13  19.11,60.66 180 top
C14  21.34,61.2 270 top
C15  24.05,67.09 0 top
C16  25.99,67.09 0 top
C17  20.94,59.09 270 top
C18  22.31,56.05 0 top
C19  18.26,56.14 180 top
C20  25.72,40.87 0 top
C21  25.45,43.32 180 top
C22  16.12,29.28 180 top
C23  25.14,76.9 180 top
C24  27.37,74.21 90 top
C25  27.69,38.77 180 top
C26  24.78,54.68 270 top
C27  24.23,56.05 0 top
C28  30.93,70.08 180 top
C29  31.48,71.48 90 top
C30  40.11,63.37 180 top
C31  40.11,62.39 180 top
C32  40.4,61.11 0 top
C33  29.5,72.97 90 top
C34  33.58,41.02 270 top
C35  32.79,41.02 270 top
C36  33.22,43.63 0 top
C37  35.32,43.61 180 top
C38  27.17,25.89 0 top
C39  32.52,21.85 90 top
C40  32.52,24.26 90 top
C41  22.7,17.69 270 top
C42  13.74,20.76 180 top
C44  27.7,39.63 180 top
C45  70.32,28.95 270 top
C46  71.43,28.95 270 top
C47  73.96,31.59 0 top
C48  77.85,26.58 90 top
C49  55.97,28.53 0 top
C50  58.39,30.65 0 top
C51  56.59,25.14 180 top
C52  60.5,26.58 90 top
C53  54.69,18.32 0 top
C54  54.58,29.84 180 top
C63  69.3,29.27 270 top
C70  71.42,33.4 0 top
CN1  66.5,7.3 0 bottom
I1  18.96,65.43 0 top
I5  32.34,56.05 0 top
I6  35.01,70.08 180 top
I7  38.46,65.06 180 top
IC1  19.04,70.58 180 top
IC2  35.77,41.19 0 top
IC3  35.57,63.55 90 top
IC4  19.96,23.9 180 top
IC9  28.29,42.16 180 top
L1  61.56,22.76 90 top
L2  20.99,65.19 270 top
L3  24.05,67.92 0 top
L4  74.76,25.48 0 top
L5  20.55,61.19 270 top
MISO2  4.9,34.6 90 bottom
MOSI2  3,34.6 90 bottom
NSS2  8.72,34.57 0 bottom
PA8  3,28.57 90 bottom
PA11  4.82,28.58 90 bottom
PA12  6.73,28.57 90 bottom
PB7  19.06,12.38 0 bottom
PB8  20.94,12.41 0 bottom
PB9  22.74,12.38 0 bottom
PC13  29.43,15.55 270 bottom
PC14  29.43,17.44 0 bottom
PC15  29.43,19.3 90 bottom
Q1  25.24,74.51 270 top
Q2  30.13,23.15 90 top
R1  16.74,56.99 270 top
R2  34.74,56.05 0 top
R3  49.36,35.3 180 top
R4  60.38,40.7 270 top
R5  19.63,30.23 270 top
R6  28.61,30.12 180 top
R7  28.62,29.26 180 top
R8  77.97,28.74 0 top
R9  77.97,29.93 180 top
R10  56,27.32 180 top
R11  61.35,28.22 180 top
R12  55.97,26.14 0 top
R13  59.19,25.65 270 top
R14  58.84,18.47 270 top
R15  57.31,19.17 180 top
R16  28.63,27.5 180 top
R17  28.62,28.37 180 top
R18  27.45,23.4 270 top
R19  20.7,17.18 270 top
R20  20.16,15.77 0 top
R21  25.33,16.25 90 top
R22  77.23,32.97 180 top
R23  24.56,31.04 270 top
R24  23.75,31.04 270 top
R25  55.9,33.13 0 top
S1  19.49,57.32 270 top
S2  28.06,71.37 270 top
SCK2  6.83,34.58 90 bottom
SV2  9.16,18.07 270 top
SV3  57.15,51.26 180 top
SWCLK  15.3,23.99 270 bottom
SWIO  13.47,23.99 90 bottom
TP1  50.9,29.8 0 top
TP2  50.9,18.4 0 top
TP3  64.6,18.4 0 top
TP4  66.6,32.6 0 top
TP5  66.6,23.9 0 top
TP6  81.3,23.9 0 top
TP7  81.3,32.6 0 top
TP8  40.7,47.7 0 top
TP9  15,47.7 0 top
TP10  40.7,79.4 0 top
TP11  15,79.4 0 top
TP12  27.76,77.24 0 top
TP13  31.23,77.2 0 top
TP14  29.52,74.96 0 top
TP15  53,12.92 0 bottom
TP17  64.6,29.8 0 top
TR1  57.87,39.41 180 top
TR2  48.12,37.91 90 top
TR3  62.58,38.33 90 top
TR6  46.33,34.27 270 top
U1  73.41,29.2 270 top
U2  57.41,22.09 180 top
VBAT  25.1,20.61 0 bottom

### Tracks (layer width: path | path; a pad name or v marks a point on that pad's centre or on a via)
5VB_EN  (via drill 0.35, 0.41)
  Top 0.203: IC4.42 19.71,20.77 19.9,20.96 20.62,20.96 20.9,21.24 v20.9,21.7 | U1.2 75.61,29.45 v75.7,29.54 | R22.2 v75.7,32.97
  Bottom 0.203: v20.9,21.7 21.28,22.08 27.97,22.08 29.36,23.47 29.36,32.74 30.24,33.62 42.74,33.62 43.76,34.64 75.01,34.64 75.7,33.95 v75.7,32.97 v75.7,29.54
+3V1
  Top 0.203: C5.1 23.22,68.76 22.7,69.28 IC1.2
+3V2
  Top 0.203: IC1.4 22.38,70.58 23.54,71.74 C6.1
+3V3  (via drill 0.35, 0.41)  (1 unrouted)
  Top 0.203: IC1.3 22.79,69.93 23.09,69.63 C4.1 C3.1 23.49,70.86 23.7,71.07 25.27,71.07 v25.51,70.83 v25.51,70.82 | IC1.24 18.39,66.8 17.94,66.35 C1.1 C2.1 15.67,66.35 15.43,66.11 15.43,64.63 15.74,64.32 v16.13,64.32 | IC2.5 35.77,41.75 35.57,41.55 33.6,41.55 C34.1 C35.1 32.48,41.57 32.09,41.96 v32.09,42.58 | IC1.14 16.72,73.92 C7.1 16.09,74.83 15.78,75.14 v15.78,76.24 | U2.6 55.53,23.09 | IC9.5 28.25,40.82 C44.1 C25.1 29.27,38.77 v29.29,38.75 | IC4.24 17.21,28.74 C22.1 v16.67,30.15 | IC4.9 25.39,25.15 26.13,25.89 C38.1 26.62,25.3 v26.05,24.73 | IC4.48 C41.1 23.27,18.24 v23.64,17.87 | IC4.36 14.52,21.15 14.29,20.92 C42.1 14.33,20.72 v14.33,19.85 | R21.2 v24.38,16.8 v24.37,16.81
  Top 0.254: 55.53,23.09 55.12,23.5
  Top 0.305: 55.12,27.29 R10.2
  Top 0.406: 55.12,23.5 R12.1
  Top 0.508: TR2.8 46.63,43.38 TR2.7 | 47.09,41.73 47.36,41.46 46.98,41.09 TR2.10
  Top 0.813: 53.23,32.6 53.22,32.61 v53.22,32.93 v53.23,32.92 v53.23,31.78
  Top 1.016: v42.06,41.31 v43.29,41.31 43.3,41.33 46.61,41.33 TR2.10 46.85,43.16 46.63,43.38 | R12.1 55.12,27.29 | R10.2 55.15,28.5 C49.1 C54.1 55.94,30.65 C50.1 R25.2 | R25.1 53.44,33.13 v53.23,32.92
  Route15 0.203: v29.29,38.75 30.49,38.75 32.01,40.27 32.01,42.65 32.09,42.73 32.09,43.09
  Route15 0.813: 52.71,32.93 49.44,32.93 48.94,33.43 | 52.71,32.93 v53.22,32.93 | 52.71,32.93 53.23,32.41 v53.23,31.78
  Route15 1.016: 45.36,33.43 44.08,34.71 44.08,40.52 v43.29,41.31 v42.06,41.31 33.35,41.31 v32.08,42.58 v32.09,42.58 32.09,43.09 32.09,48.2 30.92,49.37 24.64,49.37 23.88,50.12 23.88,70.54 24.17,70.83 v25.5,70.83 v25.51,70.82 | 45.36,33.43 48.94,33.43 | v25.58,30.13 25.58,32.26 26.75,33.43 45.36,33.43
  pour Route15 (isolate 0.406): 25.78,73.22 16.5,73.22 16.5,77 15,77 15,63.55 25.78,63.55
  pour Route15: 11.5,31 27.5,31 28.5,30 28.5,16 27.5,15 11.5,15 10.5,16 10.5,30
+3V4
  Top 0.203: IC1.25 19.04,66.2 18.27,65.43 I1.1 C9.1 C8.1
+5V  (via drill 0.35)
  Top 0.203: R8.2 79.51,28.74 79.95,29.18 79.95,31.82 79.48,32.29 71.97,32.29 71.43,31.75 C46.1
  Top 0.254: U1.7 72.58,29.8
  Top 0.305: C63.1 70.3,29.82 C45.1
  Top 0.508: TR1.7 52.41,38.35 | 52.41,38.35 52.41,38 | 52.41,38 TR1.8 | 52.41,38 54.7,38 TR1.10 54.48,38.35 52.41,38.35
  Top 0.61: 72.58,29.8 C46.1
  Top 0.813: C45.1 C46.1
  Top 1.016: TR1.10 54.7,35.88 v54.71,35.86 v53.6,35.86 | C45.1 v70.32,31.73 v70.31,31.74 C70.1
  Route15 1.016: v70.31,30.83 v70.31,31.74 70.31,34.64 69.09,35.86 v54.71,35.86 v53.6,35.86
AMP_3VEN  (via drill 0.35)
  Top 0.203: v19.26,22.5 18.8,22.04 18.8,20.97 18.71,20.88 IC4.40 | v42.47,35.22 TR6.2
  Bottom 0.203: v19.26,22.5 19.72,22.96 27.56,22.96 28.48,23.88 28.48,33.12 29.92,34.56 42.22,34.56 42.47,34.81 v42.47,35.22
AMP_5VEN  (via drill 0.35)
  Top 0.203: TR3.2 v60.9,37.38 | IC4.41 19.21,21.25 19.66,21.7 v19.88,21.7
  Bottom 0.203: v60.9,37.38 60.26,36.74 52.31,36.74 50.65,35.08 43.52,35.08 42.53,34.09 30.06,34.09 28.93,32.96 28.93,23.68 27.77,22.52 20.55,22.52 19.88,21.85 v19.88,21.7
AMPIN
  Top 0.42: C18.2 C27.1
AMPPWR  (via drill 0.35)
  Top 0.203: v48.09,44.66 v48.1,44.67 48.1,44.69
  Top 0.254: TR2.9 | TR2.9 49.18,41.29 48.76,41.72 | 50.02,41.73 TR2.9
  Top 0.813: TR2.6 49.38,43.38 | 49.38,43.38 TR2.5 | TR1.5 52.41,40.62 | TR1.6 52.41,40.62 | TR1.9 54.63,40.62 52.41,40.62 | 52.41,40.62 52.37,40.66 49.81,40.66 49.18,41.29 | TR2.9 49.39,43.37 49.38,43.38 | v39.55,58.94 v39.55,59.96 C32.1 C31.2 C30.2 I7.1
  Top 1.016: 49.38,43.38 49.32,43.44 v49.32,44.69 48.1,44.69
  Route2 0.813: v39.55,58.94 v39.55,59.96
  Route15 1.016: v39.55,59.96 v39.55,58.95 | 48.09,44.69 v49.32,44.69 41.96,44.69 40.59,46.06 40.59,57.9 v39.55,58.94
C_UART_RX
  Top 0.203: R6.2 27.61,30.12 24.64,27.14 22.88,27.14 22.71,27.31 IC4.13
C_UART_TX
  Top 0.203: IC4.12 24.82,26.65 27.43,29.26 R7.2
CP_DIO_1  (via drill 0.35)
  Top 0.203: v30.73,27.5 R16.1
  Bottom 0.203: v30.73,27.5 31,27.23 31,13.54 30.43,12.97 26.14,12.97 25.51,12.34 25.51,8.29 CN1.42
CP_DIO_2  (via drill 0.35)
  Top 0.203: v30.04,28.36 R17.1
  Bottom 0.203: CN1.43 25.05,9.85 25.05,12.56 25.97,13.48 30.24,13.48 30.55,13.79 30.55,26.64 30.04,27.15 v30.04,28.36
CP_UART_RX  (via drill 0.35)
  Top 0.203: v30.05,30.12 R6.1
  Bottom 0.203: CN1.40 27.49,8.31 27.49,11.56 27.91,11.98 30.72,11.98 31.97,13.24 31.97,29.39 31.24,30.12 v30.05,30.12
CP_UART_TX  (via drill 0.35)
  Top 0.203: v30.73,29.25 R7.1
  Bottom 0.203: CN1.41 27.01,9.81 27.01,11.75 27.73,12.47 30.56,12.47 31.49,13.4 31.49,28.49 v30.73,29.25
CW_KEY  (via drill 0.35)
  Top 0.203: IC9.1 29.24,42.46 v29.25,42.45 | IC4.38 17.71,21.21 17.98,21.48 17.98,23.61 18.76,24.39 v18.76,24.47
  Bottom 0.203: v18.76,24.47 19.14,24.47 19.77,23.84 27.17,23.84 27.6,24.27 27.6,41.58 28.47,42.45 v29.25,42.45
DIO0  (via drill 0.35)
  Top 0.203: IC1.8 20.99,75.44 v21.14,75.59 | IC4.19 19.71,26.02 20.36,25.37 v20.9,25.37
  Bottom 0.203: v21.14,75.59 21.14,74.48 17.86,71.2 17.86,47.01 18.53,46.34 22.2,46.34 22.96,45.57 22.96,29.34 21.65,28.04 21.65,25.62 21.4,25.37 v20.9,25.37
DIO1  (via drill 0.35)
  Top 0.203: IC1.9 20.34,75.35 v20.14,75.55 | IC4.18 20.21,26.63 20.49,26.35 v20.89,26.35
  Bottom 0.203: v20.14,75.55 20.14,74.17 17.42,71.45 17.42,46.76 18.31,45.87 22.02,45.87 22.51,45.38 22.51,29.47 21.24,28.2 21.24,26.68 20.91,26.35 v20.89,26.35
DIO2  (via drill 0.35)
  Top 0.203: IC1.10 19.69,74.46 19.07,75.08 v19.07,75.59 | v17.12,31.41 18.21,30.32 IC4.22
  Bottom 0.203: v19.07,75.59 18.82,75.84 17.79,75.84 16.9,74.95 10.9,74.95 10.29,74.34 10.29,41.11 11.23,40.17 16.52,40.17 17.12,39.57 v17.12,31.41
GND  (via drill 0.35, 0.8 pad 1.6)
  Top 0.203: U2.2 57.91,21.59 U2.11 | IC4.23 v17.71,26.36 | IC4.8 21.97,24.65 v21.86,24.54 v21.85,24.53 21.85,21.41 22.21,21.05 IC4.47 | v17.28,21.84 17.09,21.65 IC4.35 | R20.1 18.82,15.78 v18.69,15.65 | U2.3 59.52,22.09 59.65,21.96 59.65,19.75 v60.16,19.24
  Top 0.254: 19.69,69.93 IC1.29 | IC1.26 19.69,66.56 v19.8,66.45
  Top 0.305: IC1.23 17.74,69.05 | 17.74,69.05 17.74,69.28 | 17.74,69.28 IC1.29 | IC1.22 17.09,68.63 17.74,69.28 | IC1.21 17.32,68.63 17.74,69.05 | IC1.26 19.69,69.93 | IC1.15 17.75,72.53 18.78,71.5
  other vias: 76.42,31.37 77.41,31.37 78.42,31.37 23.43,73.65 12,57.5 12,58.5 12,59.5 12,60.5 12,61.5 12,56.5 12,55.5 12,54.5 12,53.5 12,52.5 12,51.5 12,50.5 12,49.5 12,48.5 12,47.5 13,47.75 16.7,47.75 42,47.5 43,47.5 43.75,48.75 43.75,49.75 43.75,50.75 43.75,51.75 43.75,52.75 43.75,53.75 43.75,54.75 43.75,55.75 43.75,56.75 43.75,57.75 43.75,58.75 43.75,59.75 43.75,66.75 43.75,67.75 43.75,68.75 43.75,69.75 43.75,70.75 43.75,71.75 43.75,60.75 43.75,61.75 43.75,62.75 43.75,63.75 43.75,64.75 43.75,65.75 18.75,79.5 17.75,79.5 16.75,79.5 13.75,79.5 24.75,79.5 23.75,79.5 22.75,79.5 21.75,79.5 20.75,79.5 19.75,79.5 26.75,79.5 25.75,79.5 36.64,79.5 35.53,79.51 34.4,79.5 33.29,79.5 32.25,79.51 43.75,72.75 43.75,73.75 43.75,74.75 43.75,75.75 43.75,76.75 43.75,77.75 42.75,79.5 38.75,79.5 37.75,79.5 43.75,78.75 43.75,79.75 12,68.5 12,69.5 12,70.5 12,71.5 12,72.5 12,73.5 12,62.5 12,63.5 12,64.5 12,65.5 12,66.5 12,67.5 12,76.5 12,77.5 12,78.5 12.75,79.5 11.75,79.5 34.12,62.12 30.25,63.62 30.25,62.62 30.25,64.62 31.12,62.12 32.12,62.12 33.12,62.12 31.12,65 32.12,65 33.12,65 34.12,65 33.12,66 32.12,66 31.12,66 33.12,61.12 32.12,61.12 31.12,61.12 29.25,63.62 29.25,62.62 29.25,64.62 30.25,65.62 29.25,65.62 30.25,61.62 29.25,61.62 31.12,67 32.12,67 33.12,67 30.25,66.62 29.25,66.62 29.25,60.62 30.25,60.62 31.12,60.12 32.12,60.12 33.12,60.12 23.62,47.75 22.62,47.75 20.57,47.74 39.27,47.5 35.88,47.5 34.88,47.5 33.88,47.5 24.62,47.75 25.62,47.75 26.62,47.75 27.62,47.75 28.62,47.75 29.62,47.75 30.62,47.75 28.25,63.62 28.25,62.62 28.25,64.62 28.25,65.62 28.25,61.62 28.25,66.62 28.25,60.62 18.55,47.71 37.52,47.5 41.75,77.25 40.25,77.25 38.75,77.25 37.25,77.25 35.75,77.25 34.25,77.25 32.75,77.25 32.75,74.25 32.75,75.75 34.25,75.75 34.25,74.25 34.25,72.75 35.75,72.75 37.25,72.75 37.25,74.25 35.75,74.25 35.75,75.75 37.25,75.75 38.75,75.75 40.25,75.75 41.75,75.75 38.75,74.25 38.75,72.75 38.75,71.25 38.75,69.75 40.25,69.75 40.25,71.25 40.25,72.75 40.25,74.25 41.75,74.25 41.75,72.75 41.75,71.25 41.75,69.75 41.75,68.25 41.75,66.75 41.75,65.25 40.25,66.75 40.25,68.25 23,77.25 21.5,77.25 20,77.25 18.5,77.25 17,77.25 14,77.25 14,75.75 14,73.5 30.64,72.74 32.75,72.75 16.25,49.5 16.25,51 16.25,52.5 16.25,54 16.25,59.25 16.25,60.75 16.25,62.25 25.25,59.25 25.25,60.75 25.25,62.25 25.25,63.75 25.25,65.25 26.75,65.25 26.75,63.75 26.75,62.25 26.75,60.75 26.75,59.25 28.25,59.25 30.5,68.25 29,68.25 26.75,68.25 26.75,69.75 25.25,52.5 26.75,52.5 28.25,52.5 29.75,52.5 31.25,52.5 32.75,52.5 34.25,52.5 35.75,52.5 35.75,51 35.75,49.5 34.25,49.5 34.25,51 32.75,51 31.25,51 29.75,51 28.25,51 26.75,51 25.25,51 20.75,49.5 20.75,51 20.75,52.5 20.75,54 37.52,49.5 37.52,51 37.52,52.5 37.52,54 39.31,49.5 39.31,51 39.31,52.5 39.31,54 39.31,55.5 39.31,57 18.55,49.51 18.55,51.01 18.55,52.51 18.55,54.01 42.02,49.5 42.02,51 42.02,52.4 42.02,54 42.02,55.5 42.02,57 41.72,59.2 28.39,72.74 27.66,80.81 31.34,80.78 3.5,42 3.5,45 3.5,48 3.5,51 3.5,54 3.5,57 3.5,60 3.5,63 3.5,66 3.5,69 3.5,72 3.5,75 3.5,78 3.5,81 6.5,81 9.5,81 9.5,84 6.5,84 6.5,42 6.5,45 9.5,42 9.5,45 6.5,48 6.5,51 6.5,54 6.5,57 6.5,60 6.5,63 6.5,66 6.5,69 6.5,72 9.5,48 9.5,51 9.5,54 9.5,57 9.5,60 9.5,63 9.5,66 9.5,69 9.5,72 45.5,57 45.5,60 45.5,63 45.5,66 45.5,69 45.5,72 45.5,75 45.5,78 45.5,81 48.5,57 48.5,60 48.5,63 48.5,66 48.5,69 48.5,72 48.5,75 48.5,78 48.5,81 51.5,57 51.5,60 51.5,63 51.5,66 51.5,69 51.5,72 51.5,75 51.5,78 51.5,81 54.5,57 54.5,60 54.5,63 54.5,66 54.5,69 54.5,72 54.5,75 54.5,78 54.5,81 57.5,57 57.5,60 57.5,63 57.5,66 57.5,69 57.5,72 57.5,75 57.5,78 57.5,81 60.5,57 60.5,60 60.5,63 60.5,66 60.5,69 60.5,72 60.5,75 60.5,78 60.5,81 63.5,57 63.5,60 63.5,63 63.5,66 63.5,69 63.5,72 63.5,75 63.5,78 63.5,81 66.5,57 66.5,60 66.5,63 66.5,66 66.5,69 66.5,72 66.5,75 66.5,78 66.5,81 69.5,57 69.5,60 69.5,63 69.5,66 69.5,69 69.5,72 69.5,75 69.5,78 69.5,81 72.5,48 72.5,51 72.5,54 72.5,57 72.5,60 72.5,63 72.5,66 72.5,69 72.5,72 75.5,48 75.5,51 75.5,54 75.5,57 75.5,60 75.5,63 75.5,66 75.5,69 75.5,72 81.5,48 81.5,51 81.5,54 81.5,57 81.5,60 81.5,63 81.5,66 81.5,69 81.5,72 78.5,48 78.5,51 78.5,54 78.5,57 78.5,60 78.5,63 78.5,66 78.5,69 78.5,72 81.5,45 78.5,45 75.5,45 72.5,45 69.5,45 66.5,45 63.5,45 60.5,45 57.5,45 36.5,84 33.5,84 30.5,84 27.5,84 24.5,84 21.5,84 18.5,84 15.5,84 12.5,84 63.5,84 60.5,84 57.5,84 54.5,84 51.5,84 48.5,84 45.5,84 42.5,84 39.5,84 81.5,84 78.5,84 75.5,84 72.5,84 69.5,84 66.5,84 81.5,81 78.5,81 75.5,81 72.5,81 72.5,78 72.5,75 81.5,75 81.5,78 12.5,81 15.5,81 18.5,81 21.5,81 24.5,81 33.5,81 36.5,81 42.5,81 39.5,81 3.5,39 6.5,39 9.5,39 12.5,42 12.5,45 12.5,39 15.5,39 15.5,36 12.5,36 12.5,33 15.5,33 33.5,30 36.5,30 36.5,27 39.5,27 39.5,30 39.5,36 36.5,36 33.5,36 30.5,36 42.5,39 39.5,39 39.5,45 30.5,45 27.5,45 42.5,30 45.5,30 48.5,30 48.5,27 45.5,27 42.5,27 36.5,24 36.5,21 39.5,21 39.5,24 42.5,24 42.5,21 45.5,21 45.5,24 48.5,24 48.5,21 48.5,18 45.5,18 42.5,18 39.5,18 36.5,18 36.5,15 39.5,15 42.5,15 45.5,15 48.5,15 66.5,15 69.5,15 72.5,15 75.5,15 78.5,15 81.5,15 81.5,18 81.5,21 81.5,27 81.5,30 81.5,36 78.5,36 75.5,36 72.5,36 59.81,33.06 66.5,27 66.5,21 69.5,21 72.5,21 75.5,21 69.5,24 69.5,27 78.86,33.02 69.5,39 66.5,39 66.5,42 63.5,42 69.5,42 72.5,42 72.5,39 75.5,39 75.5,42 78.5,42 78.5,39 81.5,39 81.5,42 54.5,45 51.5,45 81.5,12 81.5,9 81.5,6 78.5,12 75.5,12 72.5,12 69.5,12 66.5,12 63.5,12 72.5,9 72.5,6 72.5,3 75.5,3 78.5,3 69.5,3 69.5,6 66.5,3 63.5,3 60.5,3 57.5,3 54.5,3 51.5,3 48.5,3 45.5,3 42.5,3 39.5,3 36.5,3 33.5,3 30.5,3 27.5,3 24.5,3 21.5,3 18.5,3 15.5,3 12.5,3 9.5,3 6.5,3 3.5,6 3.5,9 3.5,12 6.5,12 9.5,12 12.5,12 15.5,12 15.5,9 15.5,6 12.5,6 12.5,9 3.5,15 3.5,18 3.5,21 15.5,15 6.5,24 3.5,24 18.5,33 18.5,36 18.5,39 18.5,42 15.5,42 18.5,45 21.5,45 21.5,36 21.5,39 21.5,42 24.5,33 24.5,36 24.5,39 24.5,45 33.5,12 36.5,12 39.5,12 42.5,12 51.5,12 54.5,12 60.5,12 57.5,12 33.5,27 33.5,15 33.5,18 33.5,21 58.67,28.24 53.3,23.99 62.41,33.04 62.41,29.57
  pour Top (isolate 0.305): -3.5,-1 -3.5,87 88.5,87 88.5,-1
  pour Bottom (isolate 0.203): -6.5,1 -6.5,-3 -6.5,-4 -1.5,-4 91.5,-4 91.5,2 91.5,87 91.5,90 88.5,90 -6.5,90 -6.5,85
  pour Route2 (isolate 0.406): -4.5,68 -4.5,88 89.5,88 89.5,79 89.5,-2 71.5,-2 -4.5,-2 -4.5,11
  pour Route15 (isolate 0.406, rank 2): -5.5,-3 90.5,-3 90.5,15 90.5,89 -5.5,89
MISO  (via drill 0.35)
  Top 0.203: IC1.17 14.75,71.23 v14.25,70.73 | v20.1,33.15 21.21,32.04 IC4.16
  Bottom 0.203: v20.1,33.15 20.07,33.15 19.74,33.48 19.74,42.52 19.08,43.18 15.15,43.18 14.17,44.16 14.17,66.15 13.78,66.54 13.78,67.74 14.44,68.4 14.44,70.54 v14.25,70.73
MOSI  (via drill 0.35)
  Top 0.203: IC1.18 15.23,70.58 14.22,69.57 v13.69,69.57 | v19.87,32.18 20.71,31.34 IC4.17
  Bottom 0.203: v19.87,32.18 19.27,32.78 19.27,42.31 18.87,42.71 14.98,42.71 13.73,43.96 13.73,65.97 13.35,66.35 13.35,67.94 13.69,68.28 v13.69,69.57
N$1
  Top 0.42: L2.2 C11.1
N$2
  Top 0.254: L5.1 C12.1
  Top 0.42: C14.1 20.96,61.74 | 20.96,61.74 L5.1 | 20.96,61.74 20.99,61.77 C11.2
N$3
  Top 0.254: C13.1 20.53,60.66 L5.2
  Top 0.42: C14.2 20.94,60.64 | 20.94,60.64 L5.2 | C17.1 20.94,60.64
N$4
  Top 0.305: S1.6 C17.2
N$5
  Top 0.406: C15.2 C16.1
N$6
  Top 0.305: C18.1 21.22,56.05 S1.4
N$7
  Top 0.305: C19.1 19.39,56.14 19.49,56.24 S1.3
N$8
  Top 0.42: R1.2 C19.2
N$9
  Top 0.42: I5.1 C27.2 C26.1
N$10  (via drill 0.35)
  Top 0.203: S2.5 S2.5 arc-90 S2.5 | v30.46,71.27 30.46,71.21 30.12,70.87 S2.5 | C37.1 36.71,43.61 | 36.71,43.61 v36.71,43.65 | 36.71,43.61 36.72,43.6 IC2.4 36.72,41.22 36.35,40.85 35.14,40.85 34.82,40.53 IC2.1
  Route15 0.203: v36.71,43.65 38.42,45.36 38.42,68.33 35.48,71.27 v30.46,71.27
N$11  (via drill 0.35)
  Top 0.203: IC9.4 C20.2 26.27,41.79 v26.06,42 | S1.2 18.91,56.82 v18.55,57.17
  Route15 0.203: v26.06,42 23.11,42 19.53,45.58 19.53,56.33 18.69,57.17 v18.55,57.17
N$12
  Top 0.42: R2.1 I5.2
N$13
  Top 0.42: IC3.1 35.59,62.03 R2.2
N$14
  Top 0.254: IC3.3 I7.2
  Top 0.42: I6.1 IC3.3
N$15
  Top 0.42: I6.2 C28.1 C29.1
N$16
  Top 0.254: S2.4 arc90 29.8,70.08
  Top 0.42: C28.2 29.8,70.08
N$17
  Top 0.203: C33.1
  Top 0.3: S2.6 C33.1
N$18  (via drill 0.35)
  Top 0.254: TR1.3 v59.13,40.05 | v59.13,40.05 v59.14,40.04 | R4.2 60.19,40.05 v59.13,40.05 | TR1.1 v59.13,37.51 v59.14,37.5
  Bottom 0.254: v59.14,40.04 58.7,40.04 58.23,39.57 58.23,38.03 58.76,37.5 v59.14,37.5
N$19  (via drill 0.35)
  Top 0.254: TR2.3 v48.76,36.62 | v48.76,36.62 v48.75,36.62 | v46.23,36.61 46.23,37.9 TR2.1 | R3.2 48.76,35.55 v48.76,36.62
  Bottom 0.254: v48.75,36.62 48.75,37.33 48.42,37.66 46.54,37.66 46.23,37.35 v46.23,36.61
N$20  (via drill 0.35)
  Top 0.203: S2.2 v27.31,70.87 | IC2.6 34.74,42.57 v33.95,42.57 33.95,43.45 C36.2
  Route15 0.203: v27.32,70.86 v27.31,70.87 27.31,70.73 28.38,69.66 35.04,69.66 36.67,68.02 36.67,45.87 33.95,43.15 v33.95,42.57
N$22  (via drill 0.35)
  Top 0.203: TR3.3 61.53,40.91 61.07,41.37 60.56,41.37 R4.1
  Top 0.254: TR1.4 59.12,41.31 | 59.12,41.31 v59.13,41.3 | R4.1 60.15,41.31 59.12,41.31 | TR1.2 v59.13,38.77 v59.14,38.77
  Bottom 0.254: v59.13,41.3 59.7,41.3 60.09,40.91 60.09,39.1 59.76,38.77 v59.14,38.77
N$23  (via drill 0.35)
  Top 0.254: TR2.4 v50.02,36.62 | v50.02,36.62 v50.03,36.62 | v47.48,36.62 TR2.2 | R3.1 50.02,35.48 50.02,35.61 | 50.02,35.61 v50.02,36.62 | TR6.3 49.79,34.27 50.07,34.55 50.07,35.56 50.02,35.61
  Bottom 0.254: v50.03,36.62 50.03,35.99 49.69,35.65 47.8,35.65 47.48,35.97 v47.48,36.62
N$24  (via drill 0.35)
  Top 0.203: R16.2 27.07,27.5 25.22,25.65 IC4.10 22.6,25.65 v22.34,25.39 | v24.54,28.7 24.54,30.47 R23.2
  Bottom 0.203: v22.34,25.39 22.64,25.69 24.04,25.69 24.54,26.19 v24.54,28.7
N$25
  Top 0.203: IC4.20 19.21,29.26 R5.2
N$26  (via drill 0.35)
  Top 0.203: R17.2 27.29,28.37 25.07,26.15 IC4.11 22.6,26.15 v22.34,26.41 | v23.75,29.48 R24.2
  Bottom 0.203: v22.34,26.41 23.02,26.41 23.75,27.14 v23.75,29.48
N$27  (via drill 0.35)
  Top 0.203: v21.76,57.26 21.76,57.15 21.43,56.83 S1.5 | IC9.6 29.24,41.57 28.97,41.84 27.64,41.84 27.34,42.14 IC9.3 27.22,43.32 C21.1 25.76,43.55 v25.76,44.19
  Route15 0.203: v21.76,57.26 21.73,57.23 21.73,46.38 23.92,44.19 v25.76,44.19
N$28
  Top 0.203: IC4.5 26.85,23.15 R18.2 29.98,22.55 Q2.1 C39.1
N$29
  Top 0.203: IC4.6 26.86,23.65 R18.1 28.28,24.25 Q2.3 29.03,24.19 29.51,23.71 C40.1
N$30
  Top 0.254: U2.4 60.23,22.59 L1.1
N$31
  Top 0.203: R9.2 R8.1 75.09,28.74 74.88,28.95 U1.3
N$32
  Top 0.254: L4.1 73.39,25.5 U1.5 73.39,31.57 C47.1
N$33
  Top 0.254: U2.5 60.39,23.09 L1.2
N$34
  Top 0.203: U1.1 74.51,30.15 C47.2
N$35  (via drill 0.35)
  Top 0.203: IC4.1 24.84,21.15 25.09,20.9 v25.09,19.18
  Bottom 0.203: VBAT.1 v25.1,19.19 v25.09,19.18
N$36
  Top 0.203: R12.2 56.36,26.14 56.04,25.82 C51.2
N$37  (via drill 0.35)
  Top 0.203: 57.74,27.32 57.74,27.3 57.75,27.3 57.75,25.35 57.54,25.14 C51.1 57.12,25.12 v57.12,24.22 | R10.1 57.74,27.32 | R11.2 C52.2 60.17,27.46 57.88,27.46 57.74,27.32
  Top 0.254: U2.9 55.31,21.59 55.02,21.3 v55.02,20.37 v55.03,20.36
  Bottom 0.203: v55.03,20.36 55.46,20.79 56.81,20.79 57.12,21.1 v57.12,24.22
N$38
  Top 0.203: IC4.44 R19.1
N$39
  Top 0.203: R13.1 59.66,26.03 C52.1
N$40  (via drill 0.35)
  Top 0.203: R13.2 58.5,24.8 v58.11,24.41 | v55.95,19.91 U2.10
  Bottom 0.203: v58.11,24.41 58.11,21 57.02,19.91 v55.95,19.91
N$41
  Top 0.254: U2.1 58.86,19.59 R14.1
N$42  (via drill 0.35)
  Top 0.203: v28.12,19.3 27.27,19.3 26.52,20.05 26.52,21.74 25.61,22.65 IC4.4
  Bottom 0.203: PC15.1 v28.12,19.3
N$44  (via drill 0.35)
  Top 0.203: IC4.3 25.45,22.15 26.08,21.52 26.08,19.84 28.07,17.85 v28.07,17.41
  Bottom 0.203: PC14.1 29.39,17.4 v28.08,17.4 v28.07,17.41
N$45  (via drill 0.35)
  Top 0.203: IC4.2 25.28,21.65 25.6,21.33 25.6,19.67 27.34,17.93 27.34,15.79 27.58,15.55 v28.09,15.55
  Bottom 0.203: PC13.1 v28.09,15.55
N$46  (via drill 0.35)
  Top 0.203: v4.92,33.16 4.92,31.97 5.63,31.26 10.79,31.26 11.77,30.27 11.77,26.82 12.94,25.65 IC4.27
  Bottom 0.203: v4.92,33.16 4.92,34.58 MISO2.1
N$47  (via drill 0.35)
  Top 0.203: v3,33.16 3,31.52 3.76,30.76 9.87,30.76 10.1,30.76 10.71,30.76 11.35,30.12 11.35,26.61 12.8,25.15 IC4.28
  Bottom 0.203: v3,33.16 MOSI2.1
N$48  (via drill 0.35)
  Top 0.203: v6.73,27.12 6.73,27.84 7.21,28.32 9.46,28.32 9.89,27.89 9.89,23.32 10.56,22.65 IC4.33
  Bottom 0.203: PA12.1 v6.73,27.12
N$49  (via drill 0.35)
  Top 0.203: v4.83,27.14 4.83,27.93 5.66,28.76 9.69,28.76 10.33,28.12 10.33,23.57 10.75,23.15 IC4.32
  Bottom 0.203: PA11.1 v4.83,27.14
N$50  (via drill 0.35)
  Top 0.203: v3,27.15 3,28.13 4.06,29.19 9.91,29.19 10.79,28.31 10.79,26.47 12.61,24.65 IC4.29
  Bottom 0.203: v3,27.15 PA8.1
N$68  (via drill 0.35)
  Top 0.203: v6.83,33.17 6.83,32.23 7.3,31.76 10.96,31.76 12.2,30.52 12.2,27.04 13.09,26.15 IC4.26
  Bottom 0.203: v6.83,33.17 SCK2.1
N$69  (via drill 0.35)
  Top 0.203: v8.72,33.2 8.72,32.57 9.03,32.26 11.04,32.26 12.65,30.65 12.65,27.27 13.27,26.65 IC4.25
  Bottom 0.203: v8.72,33.2 NSS2.1
NSSL  (via drill 0.35)
  Top 0.203: v14.87,67.15 v14.86,67.16 14.86,69.58 15.22,69.93 IC1.19 | v21.24,34.14 22.21,33.17 IC4.14
  Bottom 0.203: 14.95,67.07 v14.87,67.15 15.04,66.98 15.04,44.61 15.5,44.15 19.49,44.15 20.71,42.93 20.71,34.67 v21.24,34.14
NTRX_EN  (via drill 0.35)
  Top 0.203: v56.53,14.86 56.53,15.51 56.76,15.74 R15.2 54.79,19.17 54.37,19.59 54.37,21.75 54.71,22.09 U2.8
  Bottom 0.203: v56.53,14.86 56.53,13.33 56.12,12.92 TP15.1
PB7  (via drill 0.35)
  Top 0.203: IC4.43 20.21,18.55 19.79,18.13 18.1,18.13 17.58,17.61 17.58,14.2 18.04,13.74 v19.07,13.74
  Bottom 0.203: PB7.1 v19.06,13.73 v19.07,13.74
PB8  (via drill 0.35)
  Top 0.203: IC4.45 21.21,18.42 21.46,18.17 21.46,14.42 20.94,13.9 v20.94,13.76
  Bottom 0.203: v20.94,13.76 PB8.1
PB9  (via drill 0.35)
  Top 0.203: IC4.46 21.71,18.62 21.94,18.39 21.94,14.52 v22.74,13.72
  Bottom 0.203: v22.74,13.72 PB9.1
PROG_BOOT0  (via drill 0.35)
  Top 0.203: R19.2 R20.2 v20.71,14.77
  Bottom 0.203: v20.71,14.77 R20.2 20.09,16.38 11.07,16.38 10.43,15.74 SV2.6 10.43,15.2 11.21,14.42 13.34,14.42 14.72,13.04 14.72,5.85 15.33,5.24 62.86,5.24 63.5,5.88 63.5,8.3 CN1.3
PROG_RST  (via drill 0.35)
  Top 0.203: IC4.7 23.02,24.15 22.59,23.72 22.59,21.25 23.85,19.99 23.85,18.79 24.61,18.04 25.68,18.04 26.05,17.67 26.05,15.93 25.82,15.7 R21.1 25.28,15.75 v24.37,15.75
  Bottom 0.203: v24.37,15.75 21.44,15.75 20.33,16.86 8.55,16.86 7.89,16.2 SV2.5 7.89,14.83 8.73,13.99 13.11,13.99 14.27,12.83 14.27,5.66 15.18,4.75 63.75,4.75 64.5,5.5 CN1.4
PROG_RX  (via drill 0.35)
  Top 0.203: IC4.31 11.38,23.65 v11.2,23.84
  Bottom 0.203: v11.2,23.84 10.43,23.07 SV2.2 10.43,20.06 9.71,19.34 6.76,19.34 6.19,18.77 6.19,14.26 6.95,13.5 12.93,13.5 13.81,12.62 13.81,5.42 14.95,4.29 64.59,4.29 65.5,5.2 65.5,8.3 CN1.1
PROG_TX  (via drill 0.35)
  Top 0.203: IC4.30 11.9,24.15 v11.19,24.86
  Bottom 0.203: v11.19,24.86 9.63,23.3 9.63,22.1 8.14,20.61 SV2.1 6.42,20.61 5.77,19.96 5.77,14.06 6.78,13.05 12.69,13.05 13.38,12.36 13.38,5.17 14.72,3.83 65.38,3.83 66.5,4.95 CN1.2
RF_RX
  Top 0.254: S2.3 28.02,70.33 28.02,70.16
  Top 0.42: 28.02,70.16 28.01,70.15 28.01,68.85 28.01,68.56 arc-90 C16.2
RFI
  Top 0.305: C15.1 L3.1
  Top 0.406: IC1.1 22.02,67.83 arc90 22.75,67.09 C15.1
RFO
  Top 0.203: I1.2 20.12,65.74 L2.1
  Top 0.42: C10.1 L2.1 IC1.28
RST_L  (via drill 0.35)
  Top 0.203: v17.8,74.79 17.8,75.56 18.57,76.33 21.55,76.33 22.02,75.86 IC1.7 | v18.02,31.85 18.71,31.16 IC4.21
  Bottom 0.203: v17.8,74.79 17.52,74.51 11.15,74.51 10.76,74.12 10.76,41.27 11.41,40.62 16.73,40.62 17.56,39.8 17.56,32.31 v18.02,31.85
RX/TX_CON  (via drill 0.35)
  Top 0.203: IC2.3 v36.72,38.32 | IC4.39 18.21,21.01 18.39,21.19 18.39,22.98 v18.81,23.4
  Bottom 0.203: v36.72,38.32 36.72,38.26 36.29,37.83 28.93,37.83 28.05,36.95 28.05,24.09 27.36,23.4 v18.81,23.4
SCK  (via drill 0.35)
  Top 0.203: IC1.16 v14.24,71.88 | v21.21,33.11 21.71,32.61 IC4.15
  Bottom 0.203: 21.21,33.21 v21.21,33.11 20.24,34.08 20.24,42.68 19.26,43.66 15.34,43.66 14.61,44.39 14.61,66.35 14.2,66.76 14.2,67.53 15,68.33 15,71.42 14.54,71.88 v14.24,71.88
SWCLK  (via drill 0.35)
  Top 0.203: IC4.37 17.21,18.91 16.4,18.1 15.4,18.1 v15.37,18.13
  Bottom 0.203: v15.37,18.13 15.3,18.2 SWCLK.1
SWIO  (via drill 0.35)
  Top 0.203: IC4.34 14.03,22.15 v13.78,21.9
  Bottom 0.203: SWIO.1 13.47,22.21 v13.78,21.9
TOANT
  Top 0.406: TP14.1 29.5,74.94 C33.2
UNREG1  (via drill 0.35, 0.41)
  Top 0.203: U1.4 | 76.11,27.4 L4.2
  Top 0.254: U1.4 74.32,28.18
  Top 0.26: U2.7 54.33,22.59
  Top 0.305: 74.32,28.18 74.85,27.65 v75.49,27.65 75.86,27.65 76.11,27.4 | C53.1 53.84,22.1 54.33,22.59
  Top 0.406: C53.1 53.84,15.51 53.88,15.51 | 53.88,15.51 v53.88,14.97 | 53.88,15.51 54.42,15.51 v54.67,15.77
  Top 1.016: L4.2 76.36,25.73 C48.1 v77.85,24.39 v77.84,24.38 v77.84,23.33
  Route15 1.016: CN1.24 CN1.23 44.5,10.73 45.16,11.39 49.18,11.39 49.9,12.11 49.9,13.87 51,14.97 v53.88,14.97 v54.67,15.77 55.53,16.62 75.3,16.62 77.84,19.16 v77.84,23.33 77.84,24.91
XTA
  Top 0.203: IC1.5 22.38,71.23 23.52,72.37 25.32,72.37 25.89,72.94 Q1.3 C24.1
XTB
  Top 0.203: IC1.6 22.42,71.88 22.74,72.2 22.74,74.9 23.2,75.36 Q1.1 C23.2

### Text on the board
tPlace: RX | TX | U2 | GND | 3V3 | RST | B0

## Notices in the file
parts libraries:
SparkFun-PowerSymbols: Licensing: Creative Commons ShareAlike 4.0 International - https://creativecommons.org/licenses/by-sa/4.0
